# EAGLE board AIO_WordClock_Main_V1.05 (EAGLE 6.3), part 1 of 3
PROJECT_AUTHOR: Carsten Wille; PROJECT_COPYRIGHT: (c) 11/2012; PROJECT_NAME: WordClock; PROJECT_PCB_NO: PCB#201211001; PROJECT_REVISION: 1.05
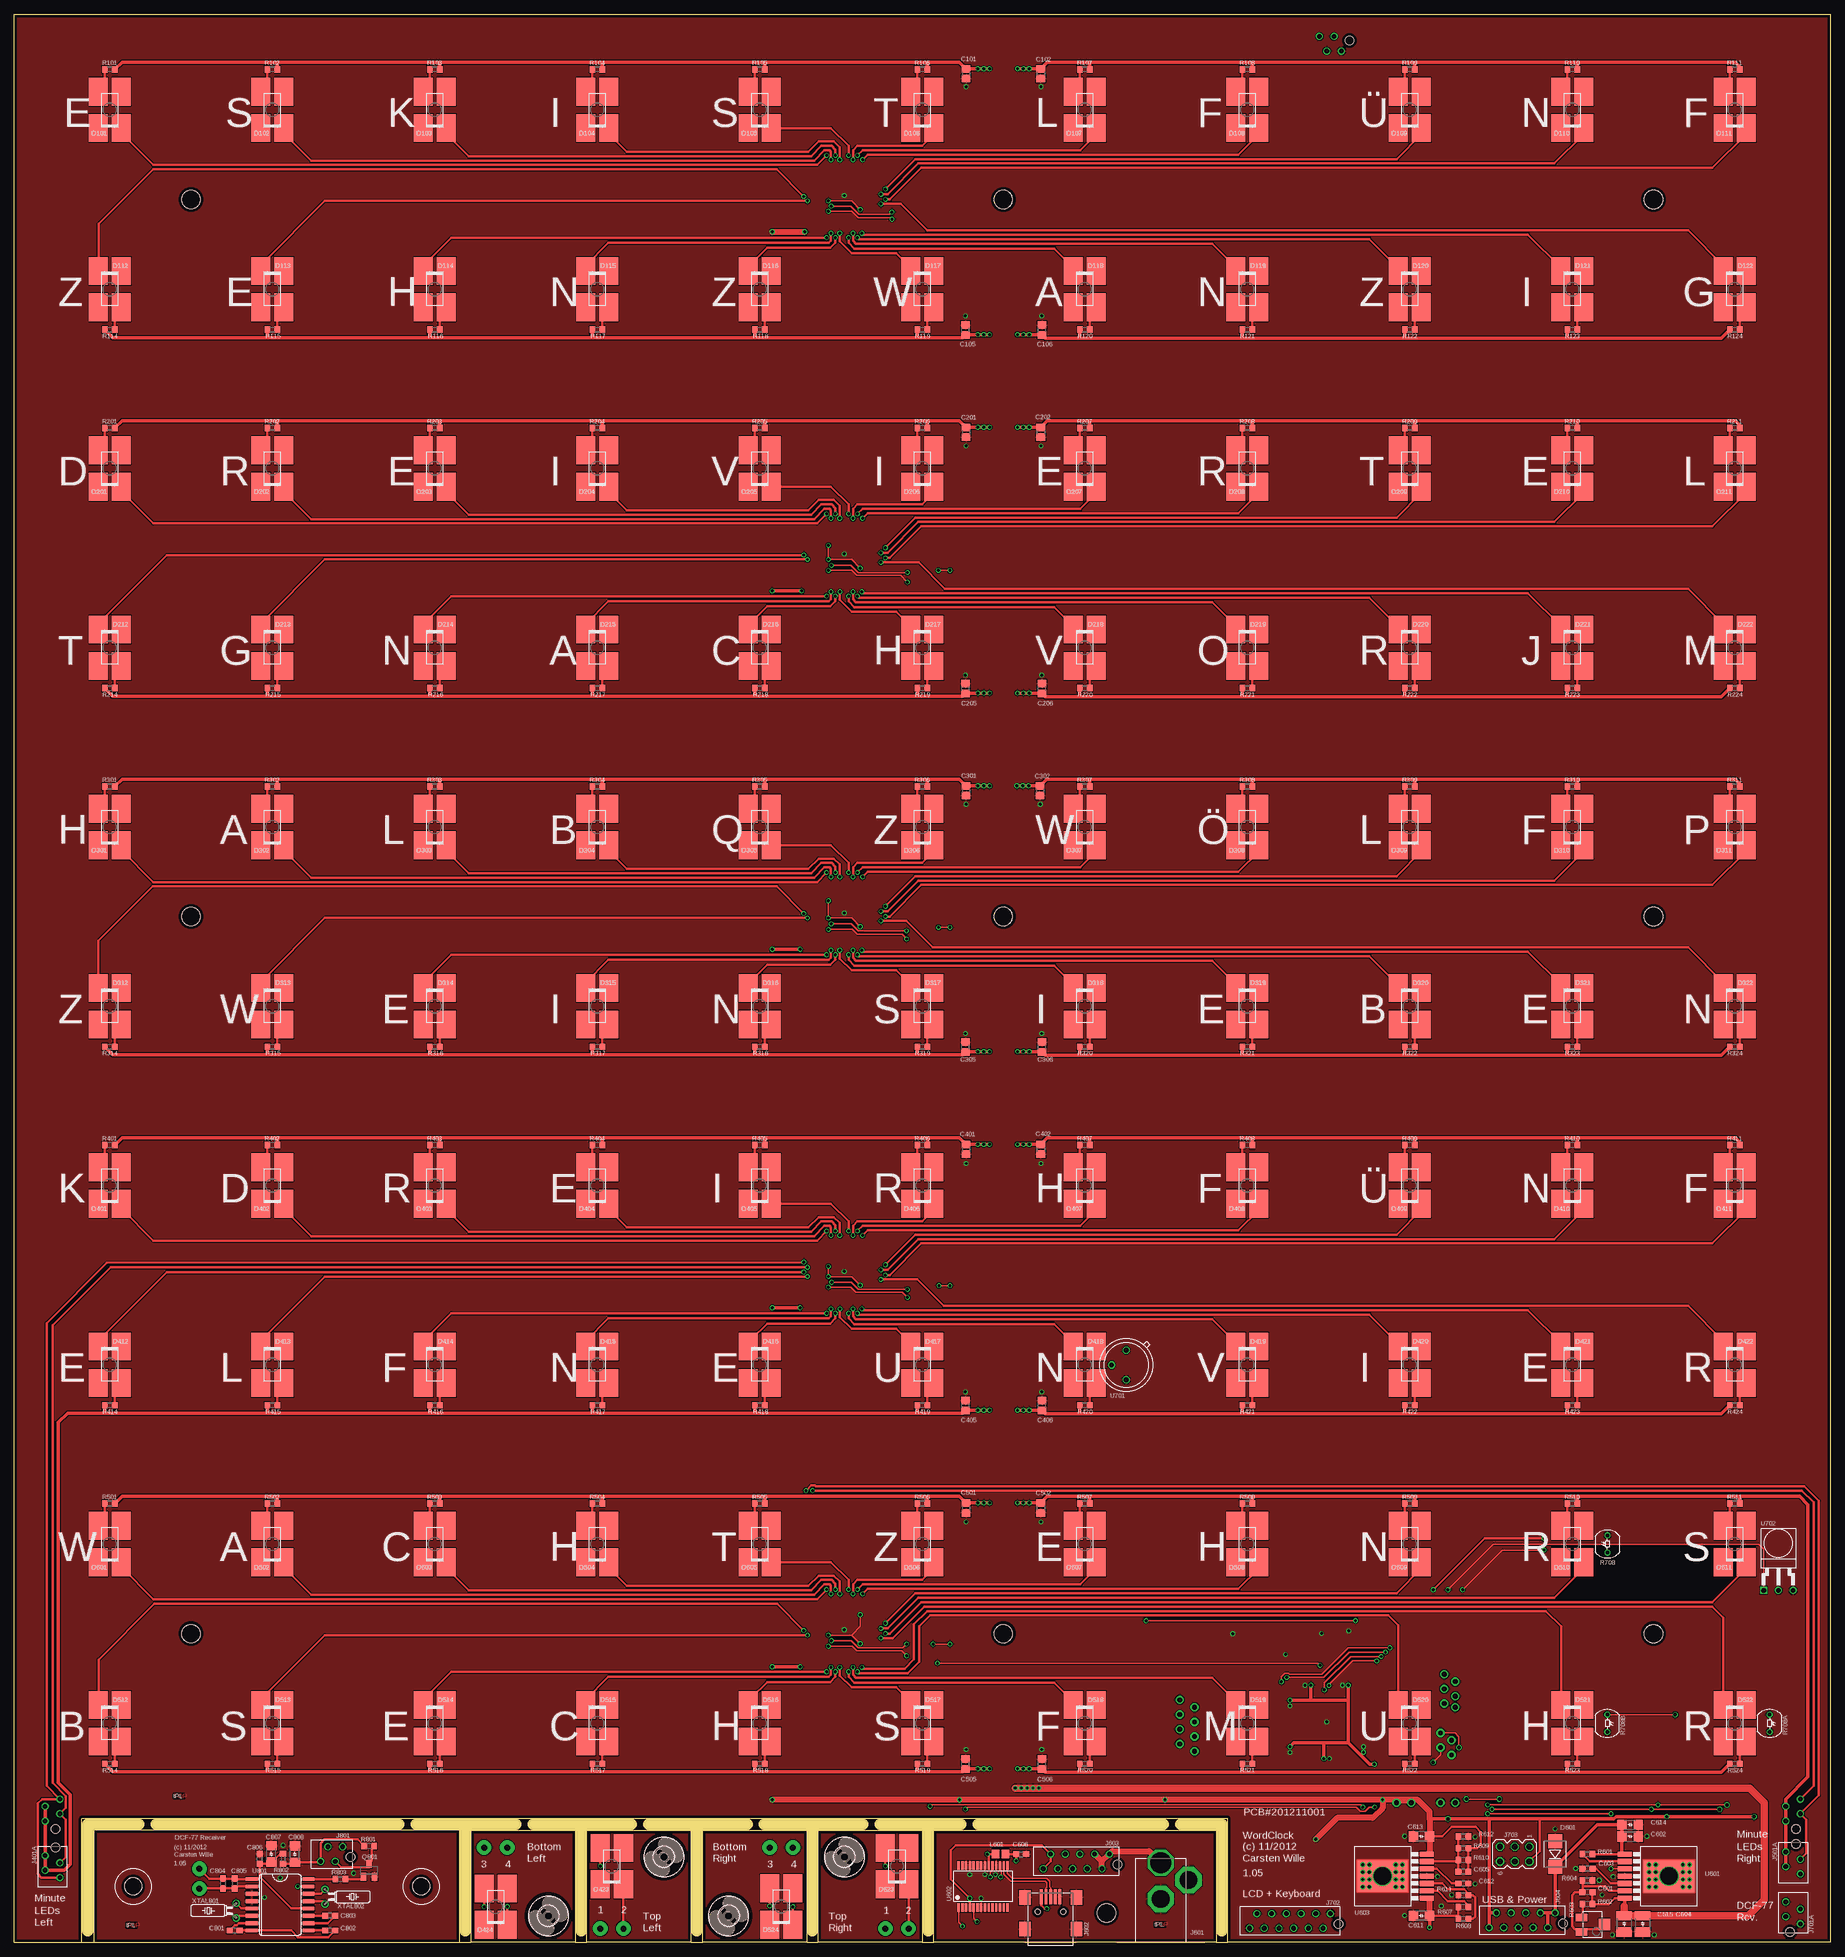
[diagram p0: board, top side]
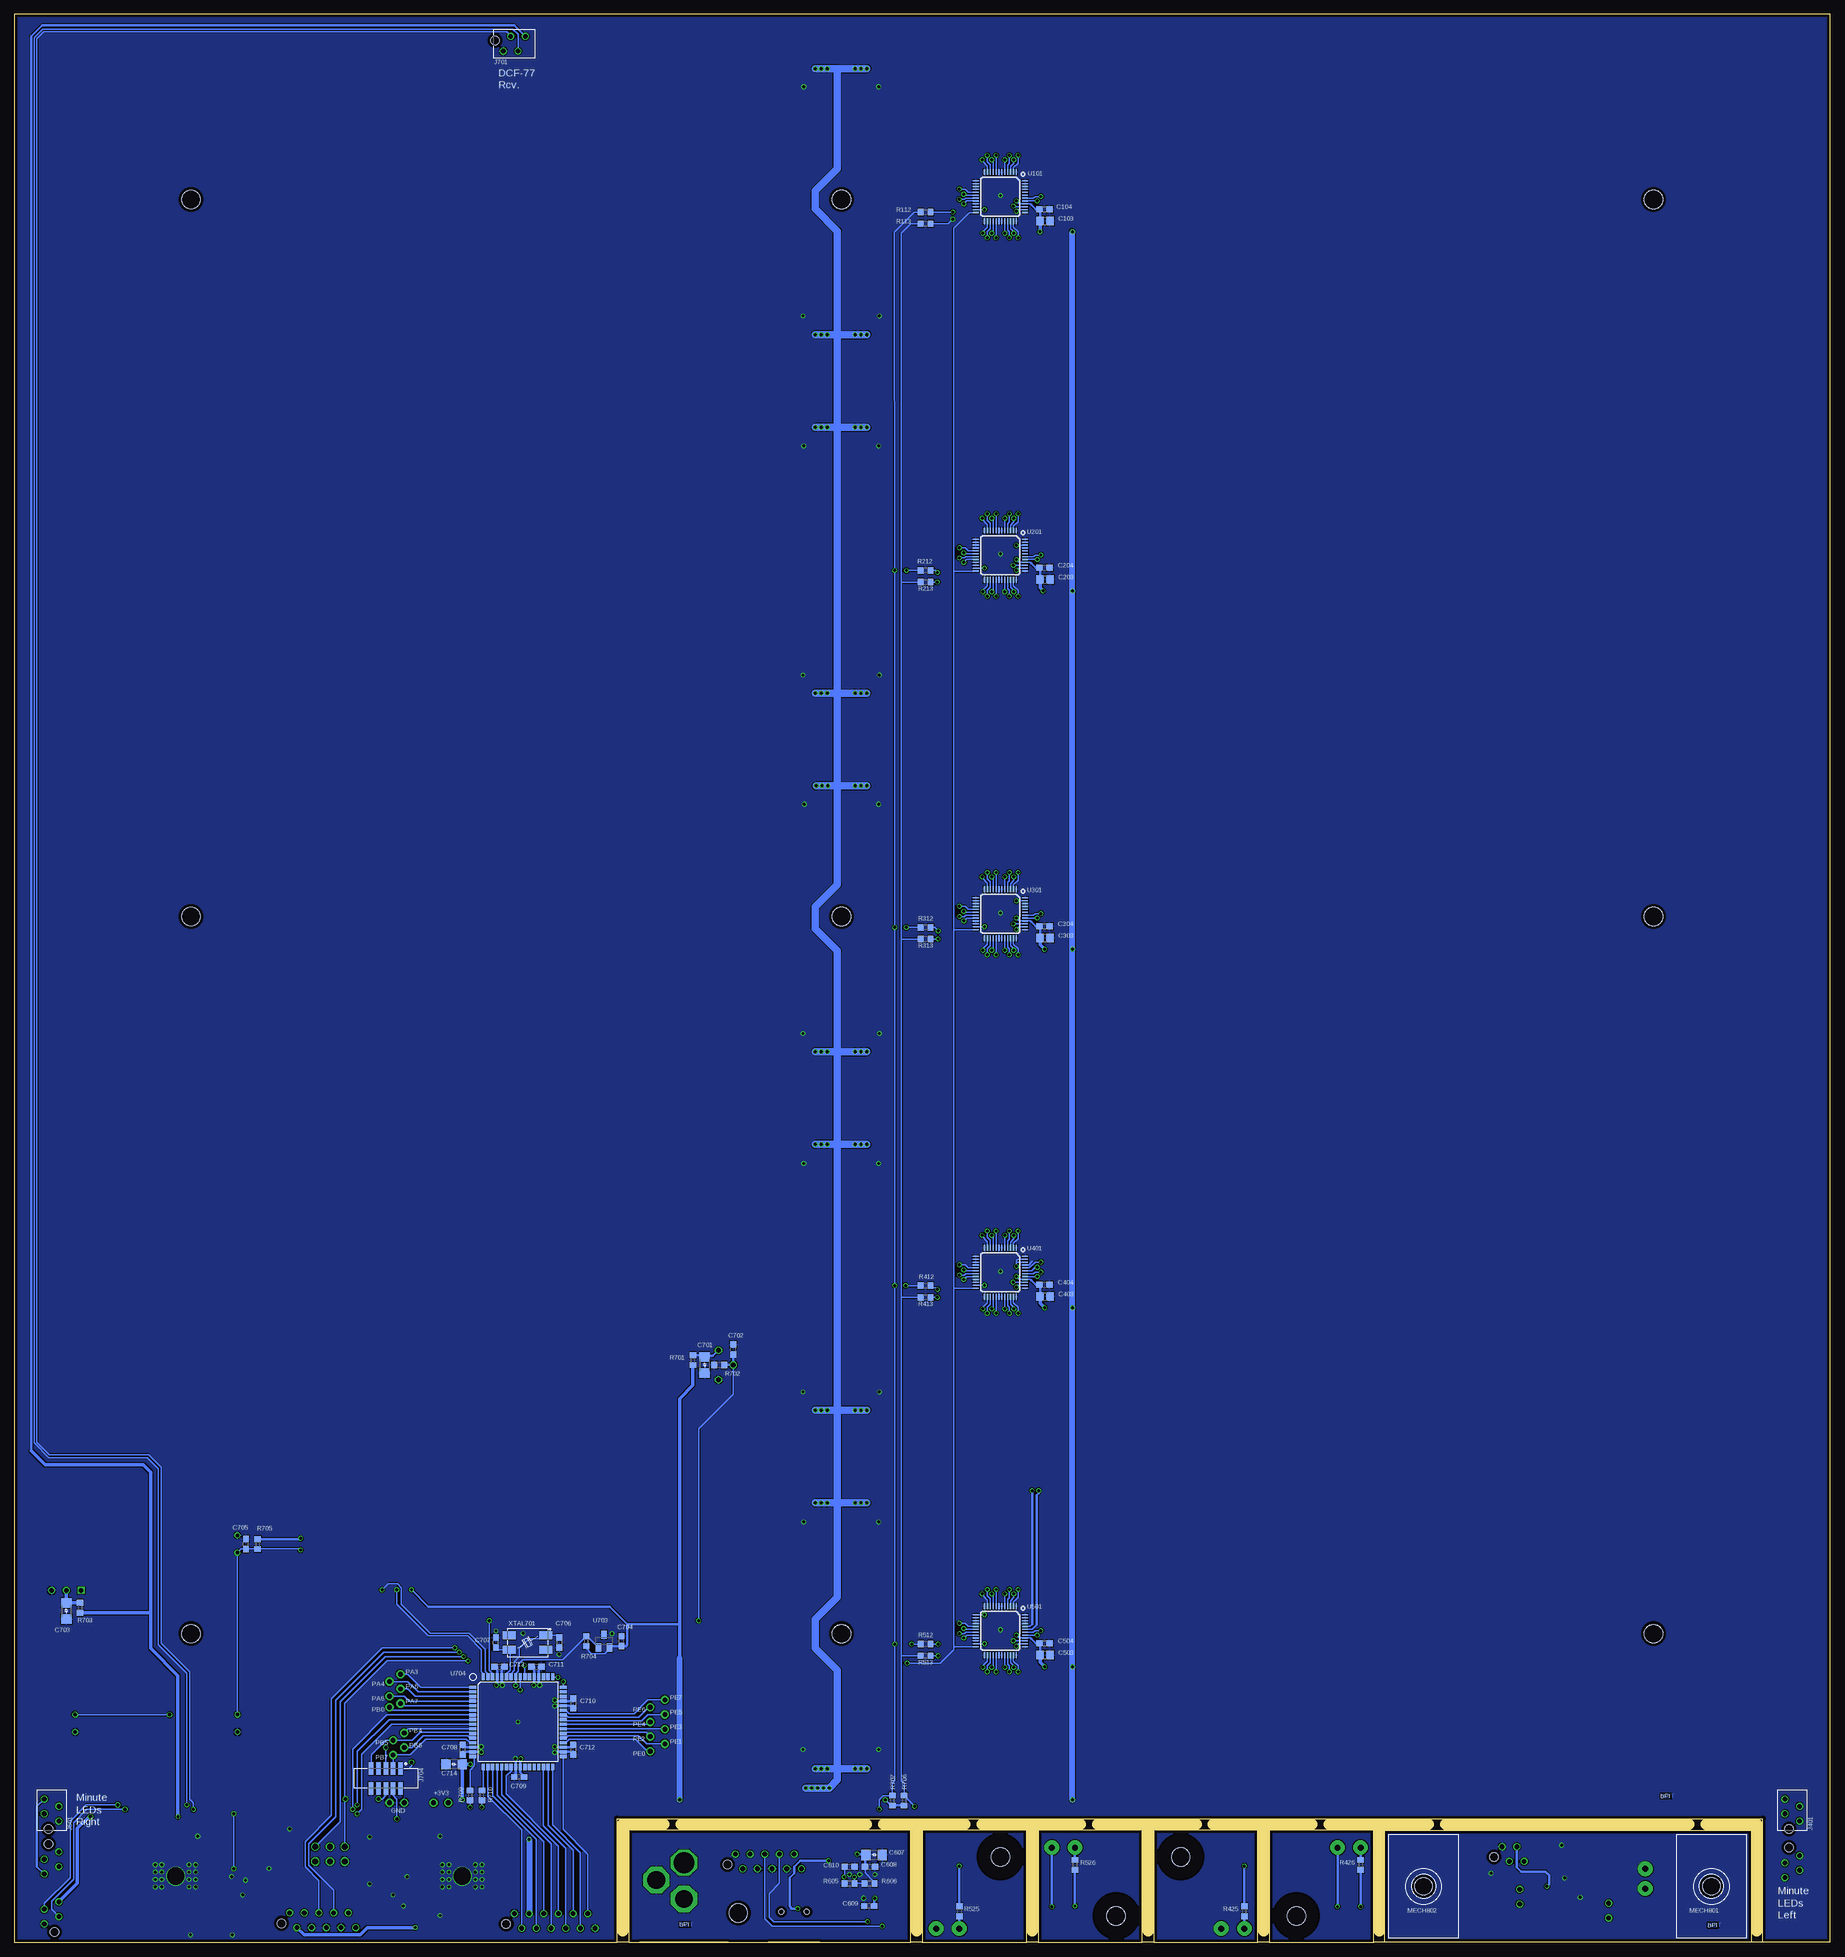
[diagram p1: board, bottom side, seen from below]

Size 314 x 333.4 mm. Coordinates in mm from the lower left corner, seen from the top.
Copper layers (1*16): Top 0.035mm / dielectric 1.5mm / Bottom 0.035mm
Design rules "leiton": minimum track width 6mil, minimum drill 12mil, track to track 6mil, track to pad 6mil, pad to pad 6mil, via to via 6mil, smd to smd 6mil, copper to edge 20mil, drill to drill 8mil, minimum pad ring 8mil, minimum via ring 6mil, stop-mask expansion 3mil, vias tented up to drill 0mil, thermal gap 8mil
Holes 3.2 mm at 188.82,5.12

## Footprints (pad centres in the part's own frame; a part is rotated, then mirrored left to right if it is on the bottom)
C0805 = smd 1.3 x 1.5: 1 -0.85,0; 2 0.85,0
C0603 = smd 1.1 x 1: 1 -0.85,0; 2 0.85,0
C1206 = smd 1.6 x 1.8: 1 -1.4,0; 2 1.4,0
C1210 = smd 1.6 x 2.7: 1 -1.4,0; 2 1.4,0
P-LCC-2 = smd 3.3 x 4.8: A -2,3.15; C 2,-3.15; NC@0 2,3.15; NC@1 -2,-3.15
SMB = smd 2.4 x 2.4: A 2.2,0; C -2.2,0
3,2 = hole 3.2: 0,0
MICRO-MATCH-4 = drill 0.8: 1 -1.905,-1.27; 2 -0.635,1.27; 3 0.635,-1.27; 4 1.905,1.27 | hole 1.5: -3.305,0.53
RAPC722X = drill 3.556 pad 4.572 octagon: 1 0,13.741 | drill 3.048 pad 4.572 octagon: 2 0,7.493; 3 4.801,10.744
USB-MINI-B-SMD = smd 2.6 x 0.5: 1 2.6,1.6; 2 2.6,0.8; 3 2.6,0; 4 2.6,-0.8; 5 2.6,-1.6 | smd 2.5 x 2: S0 -3,4.45; S1 2.5,4.45; S2 2.5,-4.45; S3 -3,-4.45 | hole 0.9: 0,2.2; 0,-2.2
MICRO-MATCH-10 = drill 0.8: 1 -5.715,-1.27; 2 -4.445,1.27; 3 -3.175,-1.27; 4 -1.905,1.27; 5 -0.635,-1.27; 6 0.635,1.27; 7 1.905,-1.27; 8 3.175,1.27; 9 4.445,-1.27; 10 5.715,1.27 | hole 1.5: -7.115,0.53
MICRO-MATCH-12 = drill 0.8: 1 -6.985,-1.27; 2 -5.715,1.27; 3 -4.445,-1.27; 4 -3.175,1.27; 5 -1.905,-1.27; 6 -0.635,1.27; 7 0.635,-1.27; 8 1.905,1.27; 9 3.175,-1.27; 10 4.445,1.27; 11 5.715,-1.27; 12 6.985,1.27 | hole 1.5: -8.385,0.53
MA03-2 = drill 1.016: 1 -1.27,2.54 | drill 1.016 octagon: 2 1.27,2.54; 3 -1.27,0; 4 1.27,0; 5 -1.27,-2.54; 6 1.27,-2.54
FTS-105-01-L-DV = smd 0.762 x 2.159: 1 -2.54,-1.714; 2 -2.54,1.714; 3 -1.27,-1.714; 4 -1.27,1.714; 5 0,-1.714; 6 0,1.714; 7 1.27,-1.714; 8 1.27,1.714; 9 2.54,-1.714; 10 2.54,1.714
L0805 = smd 1.3 x 1.5: 1 -0.85,0; 2 0.85,0
SOCKET = hole 3: 0,0
WORDCLOCK_S = hole 3.2: 281.95,30.5; 29.05,278.5; 29.05,30.5; 281.95,278.5; 29.05,154.5; 281.95,154.5; 169.5,30.5; 169.5,154.5; 169.5,278.5
SOT23 = smd 1 x 1.4: 1 -0.95,-1.1; 2 0.95,-1.1; 3 0,1.1
R0603 = smd 1 x 1.1: 1 -0.85,0; 2 0.85,0
RTRIM3224W = smd 1.3 x 2: 1 -1.25,-1.904; 3 1.25,-1.904 | smd 2 x 2: 2 0,2.031
LDR_A90 = drill 0.6: 1 -1.5,0; 2 1.5,0
LQFP48 = smd 0.203 x 1: 1 -2.75,-4.25; 2 -2.25,-4.25; 3 -1.75,-4.25; 4 -1.25,-4.25; 5 -0.75,-4.25; 6 -0.25,-4.25; 7 0.25,-4.25; 8 0.75,-4.25; 9 1.25,-4.25; 10 1.75,-4.25; 11 2.25,-4.25; 12 2.75,-4.25; 25 2.75,4.25; 26 2.25,4.25; 27 1.75,4.25; 28 1.25,4.25; 29 0.75,4.25; 30 0.25,4.25; 31 -0.25,4.25; 32 -0.75,4.25; 33 -1.25,4.25; 34 -1.75,4.25; 35 -2.25,4.25; 36 -2.75,4.25 | smd 1 x 0.203: 13 4.25,-2.75; 14 4.25,-2.25; 15 4.25,-1.75; 16 4.25,-1.25; 17 4.25,-0.75; 18 4.25,-0.25; 19 4.25,0.25; 20 4.25,0.75; 21 4.25,1.25; 22 4.25,1.75; 23 4.25,2.25; 24 4.25,2.75; 37 -4.25,2.75; 38 -4.25,2.25; 39 -4.25,1.75; 40 -4.25,1.25; 41 -4.25,0.75; 42 -4.25,0.25; 43 -4.25,-0.25; 44 -4.25,-0.75; 45 -4.25,-1.25; 46 -4.25,-1.75; 47 -4.25,-2.25; 48 -4.25,-2.75
TO-PMOD-7HS = smd 0.89 x 2.41: 1 -3.81,-7.63; 2 -2.54,-7.63; 3 -1.27,-7.63; 4 0,-7.63; 5 1.27,-7.63; 6 2.54,-7.63; 7 3.81,-7.63 | smd 5.35 x 8.54: HS 0,0
SSOP28 = smd 0.4 x 1.5: 1 -4.225,-3.625; 2 -3.575,-3.625; 3 -2.925,-3.625; 4 -2.275,-3.625; 5 -1.625,-3.625; 6 -0.975,-3.625; 7 -0.325,-3.625; 8 0.325,-3.625; 9 0.975,-3.625; 10 1.625,-3.625; 11 2.275,-3.625; 12 2.925,-3.625; 13 3.575,-3.625; 14 4.225,-3.625; 15 4.225,3.625; 16 3.575,3.625; 17 2.925,3.625; 18 2.275,3.625; 19 1.625,3.625; 20 0.975,3.625; 21 0.325,3.625; 22 -0.325,3.625; 23 -0.975,3.625; 24 -1.625,3.625; 25 -2.275,3.625; 26 -2.925,3.625; 27 -3.575,3.625; 28 -4.225,3.625
TO-5 = drill 0.813 octagon: 1 0,-2.54; 2 2.54,0; 3 0,2.54
TSOP322 = drill 0.8 square: 1 -2.54,-2.54 | drill 0.8: 2 0,-2.54; 3 2.54,-2.54
TQFP64 = smd 1.194 x 0.559: 1 -7.8,6; 2 -7.8,5.2; 3 -7.8,4.4; 4 -7.8,3.6; 5 -7.8,2.8; 6 -7.8,2; 7 -7.8,1.2; 8 -7.8,0.4; 9 -7.8,-0.4; 10 -7.8,-1.2; 11 -7.8,-2; 12 -7.8,-2.8; 13 -7.8,-3.6; 14 -7.8,-4.4; 15 -7.8,-5.2; 16 -7.8,-6; 33 7.8,-6; 34 7.8,-5.2; 35 7.8,-4.4; 36 7.8,-3.6; 37 7.8,-2.8; 38 7.8,-2; 39 7.8,-1.2; 40 7.8,-0.4; 41 7.8,0.4; 42 7.8,1.2; 43 7.8,2; 44 7.8,2.8; 45 7.8,3.6; 46 7.8,4.4; 47 7.8,5.2; 48 7.8,6 | smd 0.559 x 1.194: 17 -6,-7.8; 18 -5.2,-7.8; 19 -4.4,-7.8; 20 -3.6,-7.8; 21 -2.8,-7.8; 22 -2,-7.8; 23 -1.2,-7.8; 24 -0.4,-7.8; 25 0.4,-7.8; 26 1.2,-7.8; 27 2,-7.8; 28 2.8,-7.8; 29 3.6,-7.8; 30 4.4,-7.8; 31 5.2,-7.8; 32 6,-7.8; 49 6,7.8; 50 5.2,7.8; 51 4.4,7.8; 52 3.6,7.8; 53 2.8,7.8; 54 2,7.8; 55 1.2,7.8; 56 0.4,7.8; 57 -0.4,7.8; 58 -1.2,7.8; 59 -2,7.8; 60 -2.8,7.8; 61 -3.6,7.8; 62 -4.4,7.8; 63 -5.2,7.8; 64 -6,7.8
SO16L = smd 0.66 x 2.032: 1 -4.445,-4.902; 2 -3.175,-4.902; 3 -1.905,-4.902; 4 -0.635,-4.902; 5 0.635,-4.902; 6 1.905,-4.902; 7 3.175,-4.902; 8 4.445,-4.902; 9 4.445,4.902; 10 3.175,4.902; 11 1.905,4.902; 12 0.635,4.902; 13 -0.635,4.902; 14 -1.905,4.902; 15 -3.175,4.902; 16 -4.445,4.902
SINGLE-PIN = drill 0.813 pad 1.422: P$1 0,0
SINGLE-PIN_BIG = drill 1.016 pad 2.54: 1 0,0
MQ = smd 2.2 x 1.4: 1 -3.15,-1.25; 2 3.15,-1.25; 3 3.15,1.25; 4 -3.15,1.25
TC26H = drill 0.813: 1 -1.27,0; 2 1.27,0

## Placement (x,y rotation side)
C101  1E-6-1U-0805  [C0805]  164.57,323.15 270 top
C102  1E-6-1U-0805  [C0805]  177.46,323.15 270 top
C103  1E-6-1U-0805  [C0805]  135.81,297.7 0 bottom
C104  1E-9-100N-0603  [C0603]  135.88,299.73 0 bottom
C105  1E-6-1U-0805  [C0805]  164.47,278.84 90 top
C106  1E-6-1U-0805  [C0805]  177.69,278.84 90 top
C201  1E-6-1U-0805  [C0805]  164.57,261.15 270 top
C202  1E-6-1U-0805  [C0805]  177.46,261.15 270 top
C203  1E-6-1U-0805  [C0805]  135.81,235.7 0 bottom
C204  1E-9-100N-0603  [C0603]  135.88,237.73 0 bottom
C205  1E-6-1U-0805  [C0805]  164.47,216.84 90 top
C206  1E-6-1U-0805  [C0805]  177.69,216.84 90 top
C301  1E-6-1U-0805  [C0805]  164.57,199.15 270 top
C302  1E-6-1U-0805  [C0805]  177.33,199.15 270 top
C303  1E-6-1U-0805  [C0805]  135.81,173.7 0 bottom
C304  1E-9-100N-0603  [C0603]  135.88,175.73 0 bottom
C305  1E-6-1U-0805  [C0805]  164.47,154.84 90 top
C306  1E-6-1U-0805  [C0805]  177.69,154.84 90 top
C401  1E-6-1U-0805  [C0805]  164.57,137.15 270 top
C402  1E-6-1U-0805  [C0805]  177.46,137.15 270 top
C403  1E-6-1U-0805  [C0805]  135.81,111.7 0 bottom
C404  1E-9-100N-0603  [C0603]  135.88,113.73 0 bottom
C405  1E-6-1U-0805  [C0805]  164.47,92.84 90 top
C406  1E-6-1U-0805  [C0805]  177.69,92.84 90 top
C501  1E-6-1U-0805  [C0805]  164.57,75.15 270 top
C502  1E-6-1U-0805  [C0805]  177.46,75.15 270 top
C503  1E-6-1U-0805  [C0805]  135.81,49.7 0 bottom
C504  1E-9-100N-0603  [C0603]  135.88,51.73 0 bottom
C505  1E-6-1U-0805  [C0805]  164.47,30.84 90 top
C506  1E-6-1U-0805  [C0805]  177.69,30.84 90 top
C601  1E-9-22N-0603  [C0603]  272.01,8.68 180 top
C602  1E-6-10U-1206  [C1206]  279.38,18.33 0 top
C603  1E-9-22N-0603  [C0603]  272.01,12.74 180 top
C604  1E-6-47U-1210  [C1210]  281.54,3.21 270 top
C605  1E-9-22N-0603  [C0603]  250.55,12.23 180 top
C606  1E-9-10N-0603  [C0603]  174.09,15.28 0 top
C607  1E-6-10U-1206  [C1206]  165.33,15.15 0 bottom
C608  1E-9-100N-0603  [C0603]  166.07,13.07 0 bottom
C609  1E-9-100N-0603  [C0603]  166.19,6.31 180 bottom
C610  1E-9-100N-0603  [C0603]  169.57,13.07 0 bottom
C611  1E-6-10U-1206  [C1206]  243.31,4.61 180 top
C612  1E-9-22N-0603  [C0603]  250.55,10.2 0 top
C613  1E-6-10U-1206  [C1206]  243.31,18.33 180 top
C614  1E-6-10U-1206  [C1206]  279.38,20.36 0 top
C615  1E-6-47U-1210  [C1210]  278.36,3.21 270 top
C701  1E-6-10U-1206  [C1206]  194.67,99.86 270 bottom
C702  1E-9-33N-0603  [C0603]  189.71,102.53 90 bottom
C703  1E-6-10U-1206  [C1206]  305.03,57.32 270 bottom
C704  1E-9-100N-0603  [C0603]  209.02,52.11 90 bottom
C705  1E-9-33N-0603  [C0603]  273.97,68.9 90 bottom
C706  1E-12-22P-0603  [C0603]  219.81,51.86 270 bottom
C707  1E-12-22P-0603  [C0603]  230.74,51.86 90 bottom
C708  1E-9-100N-0603  [C0603]  236.48,33.34 90 bottom
C709  1E-9-100N-0603  [C0603]  226.72,28.61 180 bottom
C710  1E-9-100N-0603  [C0603]  217.37,41.34 270 bottom
C711  1E-9-100N-0603  [C0603]  223.72,47.69 0 bottom
C712  1E-9-100N-0603  [C0603]  217.37,33.34 270 bottom
C713  1E-9-100N-0603  [C0603]  230.13,47.69 0 bottom
C714  1E-6-10U-1206  [C1206]  237.97,30.82 180 bottom
C801  1E-9-6.8N-0603  [C0603]  38.08,2.07 0 top
C802  1E-9-33N-0603  [C0603]  54.59,2.07 180 top
C803  1E-9-10N-0603  [C0603]  54.59,4.61 180 top
C804  1E-9-1.5N-0603  [C0603]  36.04,10.2 270 top
C805  1E-9-1.5N-0603  [C0603]  38.08,10.2 270 top
C806  1E-9-100N-0603  [C0603]  42.39,14.47 90 top
C807  1E-6-10U-1206  [C1206]  44.43,15.31 90 top
C808  1E-6-10U-1206  [C1206]  48.49,15.28 90 top
D101  TOPLED-LUW  [P-LCC-2]  16.5,316.9 0 top
D102  TOPLED-LUW  [P-LCC-2]  44.6,316.9 0 top
D103  TOPLED-LUW  [P-LCC-2]  72.7,316.9 0 top
D104  TOPLED-LUW  [P-LCC-2]  100.8,316.9 0 top
D105  TOPLED-LUW  [P-LCC-2]  128.9,316.9 0 top
D106  TOPLED-LUW  [P-LCC-2]  157,316.9 0 top
D107  TOPLED-LUW  [P-LCC-2]  185.1,316.9 0 top
D108  TOPLED-LUW  [P-LCC-2]  213.2,316.9 0 top
D109  TOPLED-LUW  [P-LCC-2]  241.3,316.9 0 top
D110  TOPLED-LUW  [P-LCC-2]  269.4,316.9 0 top
D111  TOPLED-LUW  [P-LCC-2]  297.5,316.9 0 top
D112  TOPLED-LUW  [P-LCC-2]  16.5,285.9 180 top
D113  TOPLED-LUW  [P-LCC-2]  44.6,285.9 180 top
D114  TOPLED-LUW  [P-LCC-2]  72.7,285.9 180 top
D115  TOPLED-LUW  [P-LCC-2]  100.8,285.9 180 top
D116  TOPLED-LUW  [P-LCC-2]  128.9,285.9 180 top
D117  TOPLED-LUW  [P-LCC-2]  157,285.9 180 top
D118  TOPLED-LUW  [P-LCC-2]  185.1,285.9 180 top
D119  TOPLED-LUW  [P-LCC-2]  213.2,285.9 180 top
D120  TOPLED-LUW  [P-LCC-2]  241.3,285.9 180 top
D121  TOPLED-LUW  [P-LCC-2]  269.4,285.9 180 top
D122  TOPLED-LUW  [P-LCC-2]  297.5,285.9 180 top
D201  TOPLED-LUW  [P-LCC-2]  16.5,254.9 0 top
D202  TOPLED-LUW  [P-LCC-2]  44.6,254.9 0 top
D203  TOPLED-LUW  [P-LCC-2]  72.7,254.9 0 top
D204  TOPLED-LUW  [P-LCC-2]  100.8,254.9 0 top
D205  TOPLED-LUW  [P-LCC-2]  128.9,254.9 0 top
D206  TOPLED-LUW  [P-LCC-2]  157,254.9 0 top
D207  TOPLED-LUW  [P-LCC-2]  185.1,254.9 0 top
D208  TOPLED-LUW  [P-LCC-2]  213.2,254.9 0 top
D209  TOPLED-LUW  [P-LCC-2]  241.3,254.9 0 top
D210  TOPLED-LUW  [P-LCC-2]  269.4,254.9 0 top
D211  TOPLED-LUW  [P-LCC-2]  297.5,254.9 0 top
D212  TOPLED-LUW  [P-LCC-2]  16.5,223.9 180 top
D213  TOPLED-LUW  [P-LCC-2]  44.6,223.9 180 top
D214  TOPLED-LUW  [P-LCC-2]  72.7,223.9 180 top
D215  TOPLED-LUW  [P-LCC-2]  100.8,223.9 180 top
D216  TOPLED-LUW  [P-LCC-2]  128.9,223.9 180 top
D217  TOPLED-LUW  [P-LCC-2]  157,223.9 180 top
D218  TOPLED-LUW  [P-LCC-2]  185.1,223.9 180 top
D219  TOPLED-LUW  [P-LCC-2]  213.2,223.9 180 top
D220  TOPLED-LUW  [P-LCC-2]  241.3,223.9 180 top
D221  TOPLED-LUW  [P-LCC-2]  269.4,223.9 180 top
D222  TOPLED-LUW  [P-LCC-2]  297.5,223.9 180 top
D301  TOPLED-LUW  [P-LCC-2]  16.5,192.9 0 top
D302  TOPLED-LUW  [P-LCC-2]  44.6,192.9 0 top
D303  TOPLED-LUW  [P-LCC-2]  72.7,192.9 0 top
D304  TOPLED-LUW  [P-LCC-2]  100.8,192.9 0 top
D305  TOPLED-LUW  [P-LCC-2]  128.9,192.9 0 top
D306  TOPLED-LUW  [P-LCC-2]  157,192.9 0 top
D307  TOPLED-LUW  [P-LCC-2]  185.1,192.9 0 top
D308  TOPLED-LUW  [P-LCC-2]  213.2,192.9 0 top
D309  TOPLED-LUW  [P-LCC-2]  241.3,192.9 0 top
D310  TOPLED-LUW  [P-LCC-2]  269.4,192.9 0 top
D311  TOPLED-LUW  [P-LCC-2]  297.5,192.9 0 top
D312  TOPLED-LUW  [P-LCC-2]  16.5,161.9 180 top
D313  TOPLED-LUW  [P-LCC-2]  44.6,161.9 180 top
D314  TOPLED-LUW  [P-LCC-2]  72.7,161.9 180 top
D315  TOPLED-LUW  [P-LCC-2]  100.8,161.9 180 top
D316  TOPLED-LUW  [P-LCC-2]  128.9,161.9 180 top
D317  TOPLED-LUW  [P-LCC-2]  157,161.9 180 top
D318  TOPLED-LUW  [P-LCC-2]  185.1,161.9 180 top
D319  TOPLED-LUW  [P-LCC-2]  213.2,161.9 180 top
D320  TOPLED-LUW  [P-LCC-2]  241.3,161.9 180 top
D321  TOPLED-LUW  [P-LCC-2]  269.4,161.9 180 top
D322  TOPLED-LUW  [P-LCC-2]  297.5,161.9 180 top
D401  TOPLED-LUW  [P-LCC-2]  16.5,130.9 0 top
D402  TOPLED-LUW  [P-LCC-2]  44.6,130.9 0 top
D403  TOPLED-LUW  [P-LCC-2]  72.7,130.9 0 top
D404  TOPLED-LUW  [P-LCC-2]  100.8,130.9 0 top
D405  TOPLED-LUW  [P-LCC-2]  128.9,130.9 0 top
D406  TOPLED-LUW  [P-LCC-2]  157,130.9 0 top
D407  TOPLED-LUW  [P-LCC-2]  185.1,130.9 0 top
D408  TOPLED-LUW  [P-LCC-2]  213.2,130.9 0 top
D409  TOPLED-LUW  [P-LCC-2]  241.3,130.9 0 top
D410  TOPLED-LUW  [P-LCC-2]  269.4,130.9 0 top
D411  TOPLED-LUW  [P-LCC-2]  297.5,130.9 0 top
D412  TOPLED-LUW  [P-LCC-2]  16.5,99.9 180 top
D413  TOPLED-LUW  [P-LCC-2]  44.6,99.9 180 top
D414  TOPLED-LUW  [P-LCC-2]  72.7,99.9 180 top
D415  TOPLED-LUW  [P-LCC-2]  100.8,99.9 180 top
D416  TOPLED-LUW  [P-LCC-2]  128.9,99.9 180 top
D417  TOPLED-LUW  [P-LCC-2]  157,99.9 180 top
D418  TOPLED-LUW  [P-LCC-2]  185.1,99.9 180 top
D419  TOPLED-LUW  [P-LCC-2]  213.2,99.9 180 top
D420  TOPLED-LUW  [P-LCC-2]  241.3,99.9 180 top
D421  TOPLED-LUW  [P-LCC-2]  269.4,99.9 180 top
D422  TOPLED-LUW  [P-LCC-2]  297.5,99.9 180 top
D423  TOPLED-LUW  [P-LCC-2]  103.31,13.2 0 top
D424  TOPLED-LUW  [P-LCC-2]  83.21,6.2 0 top
D501  TOPLED-LUW  [P-LCC-2]  16.5,68.9 0 top
D502  TOPLED-LUW  [P-LCC-2]  44.6,68.9 0 top
D503  TOPLED-LUW  [P-LCC-2]  72.7,68.9 0 top
D504  TOPLED-LUW  [P-LCC-2]  100.8,68.9 0 top
D505  TOPLED-LUW  [P-LCC-2]  128.9,68.9 0 top
D506  TOPLED-LUW  [P-LCC-2]  157,68.9 0 top
D507  TOPLED-LUW  [P-LCC-2]  185.1,68.9 0 top
D508  TOPLED-LUW  [P-LCC-2]  213.2,68.9 0 top
D509  TOPLED-LUW  [P-LCC-2]  241.3,68.9 0 top
D510  TOPLED-LUW  [P-LCC-2]  269.4,68.9 0 top
D511  TOPLED-LUW  [P-LCC-2]  297.5,68.9 0 top
D512  TOPLED-LUW  [P-LCC-2]  16.5,37.9 180 top
D513  TOPLED-LUW  [P-LCC-2]  44.6,37.9 180 top
D514  TOPLED-LUW  [P-LCC-2]  72.7,37.9 180 top
D515  TOPLED-LUW  [P-LCC-2]  100.8,37.9 180 top
D516  TOPLED-LUW  [P-LCC-2]  128.9,37.9 180 top
D517  TOPLED-LUW  [P-LCC-2]  157,37.9 180 top
D518  TOPLED-LUW  [P-LCC-2]  185.1,37.9 180 top
D519  TOPLED-LUW  [P-LCC-2]  213.2,37.9 180 top
D520  TOPLED-LUW  [P-LCC-2]  241.3,37.9 180 top
D521  TOPLED-LUW  [P-LCC-2]  269.4,37.9 180 top
D522  TOPLED-LUW  [P-LCC-2]  297.5,37.9 180 top
D523  TOPLED-LUW  [P-LCC-2]  152.61,13.2 0 top
D524  TOPLED-LUW  [P-LCC-2]  132.6,6.22 0 top
D601  20BQ030-SMB  [SMB]  266.42,15.28 90 top
H401  MOUNT-HOLE3.2  [3,2]  92.31,4.6 0 top
H402  MOUNT-HOLE3.2  [3,2]  112.31,14.8 0 top
H501  MOUNT-HOLE3.2  [3,2]  123.51,4.6 0 top
H502  MOUNT-HOLE3.2  [3,2]  143.51,14.8 0 top
J401  MICRO-MATCH-4  [MICRO-MATCH-4]  6.58,22.9 90 bottom
J401A  MICRO-MATCH-4  [MICRO-MATCH-4]  6.58,13.12 270 top
J501  MICRO-MATCH-4  [MICRO-MATCH-4]  307.57,22.9 90 bottom
J501A  MICRO-MATCH-4  [MICRO-MATCH-4]  307.57,13.76 270 top
J601  PWR-JACK  [RAPC722X]  198.22,0.04 0 top
J602  USB_B_MINI  [USB-MINI-B-SMD]  179.17,5.3 90 top
J603  MICRO-MATCH-10  [MICRO-MATCH-10]  183.62,14.01 180 top
J604  MICRO-MATCH-10  [MICRO-MATCH-10]  260.71,3.85 180 top
J701  MICRO-MATCH-4  [MICRO-MATCH-4]  227.56,328.33 0 bottom
J701A  MICRO-MATCH-4  [MICRO-MATCH-4]  307.57,5.12 90 top
J702  MICRO-MATCH-12  [MICRO-MATCH-12]  220.57,3.72 180 top
J703  PROG-PDI  [MA03-2]  259.44,15.28 270 top
J704  JTAG_ATMEL-50MIL  [FTS-105-01-L-DV]  249.78,28.36 180 bottom
J801  MICRO-MATCH-4  [MICRO-MATCH-4]  54.84,15.28 180 top
L601  L-1U0-0805  [L0805]  170.54,15.28 180 top
MECH801  SOCKET  [SOCKET]  20.55,9.69 0 bottom
MECH802  SOCKET  [SOCKET]  70.33,9.69 0 bottom
PCB1  PCB-WORDCLOCK-ALL-IN-ONE  [WORDCLOCK_S]  1.5,22.9 0 top
Q801  BC847  [SOT23]  61.32,12.49 0 top
R101  1E0-3,0R-0603  [R0603]  16.5,323.9 180 top
R102  1E0-3,0R-0603  [R0603]  44.6,323.9 180 top
R103  1E0-3,0R-0603  [R0603]  72.7,323.9 180 top
R104  1E0-3,0R-0603  [R0603]  100.8,323.9 180 top
R105  1E0-3,0R-0603  [R0603]  128.9,323.9 180 top
R106  1E0-3,0R-0603  [R0603]  157,323.9 180 top
R107  1E0-3,0R-0603  [R0603]  185.1,323.9 180 top
R108  1E0-3,0R-0603  [R0603]  213.2,323.9 180 top
R109  1E0-3,0R-0603  [R0603]  241.3,323.9 180 top
R110  1E0-3,0R-0603  [R0603]  269.4,323.9 180 top
R111  1E0-3,0R-0603  [R0603]  297.5,323.9 180 top
R112  1E2-330R-0603  [R0603]  156.44,299.23 0 bottom
R113  1E2-330R-0603  [R0603]  156.44,297.22 0 bottom
R114  1E0-3,0R-0603  [R0603]  16.5,278.9 180 top
R115  1E0-3,0R-0603  [R0603]  44.6,278.9 180 top
R116  1E0-3,0R-0603  [R0603]  72.7,278.9 180 top
R117  1E0-3,0R-0603  [R0603]  100.8,278.9 180 top
R118  1E0-3,0R-0603  [R0603]  128.9,278.9 180 top
R119  1E0-3,0R-0603  [R0603]  157,278.9 180 top
R120  1E0-3,0R-0603  [R0603]  185.1,278.9 180 top
R121  1E0-3,0R-0603  [R0603]  213.2,278.9 180 top
R122  1E0-3,0R-0603  [R0603]  241.3,278.9 180 top
R123  1E0-3,0R-0603  [R0603]  269.4,278.9 180 top
R124  1E0-3,0R-0603  [R0603]  297.5,278.9 180 top
R201  1E0-3,0R-0603  [R0603]  16.5,261.9 180 top
R202  1E0-3,0R-0603  [R0603]  44.6,261.9 180 top
R203  1E0-3,0R-0603  [R0603]  72.7,261.9 180 top
R204  1E0-3,0R-0603  [R0603]  100.8,261.9 180 top
R205  1E0-3,0R-0603  [R0603]  128.9,261.9 180 top
R206  1E0-3,0R-0603  [R0603]  157,261.9 180 top
R207  1E0-3,0R-0603  [R0603]  185.1,261.9 180 top
R208  1E0-3,0R-0603  [R0603]  213.2,261.9 180 top
R209  1E0-3,0R-0603  [R0603]  241.3,261.9 180 top
R210  1E0-3,0R-0603  [R0603]  269.4,261.9 180 top
R211  1E0-3,0R-0603  [R0603]  297.5,261.9 180 top
R212  1E2-330R-0603  [R0603]  156.44,237.28 0 bottom
R213  1E2-330R-0603  [R0603]  156.44,235.24 0 bottom
R214  1E0-3,0R-0603  [R0603]  16.5,216.9 180 top
R215  1E0-3,0R-0603  [R0603]  44.6,216.9 180 top
R216  1E0-3,0R-0603  [R0603]  72.7,216.9 180 top
R217  1E0-3,0R-0603  [R0603]  100.8,216.9 180 top
R218  1E0-3,0R-0603  [R0603]  128.9,216.9 180 top
R219  1E0-3,0R-0603  [R0603]  157,216.9 180 top
R220  1E0-3,0R-0603  [R0603]  185.1,216.9 180 top
R221  1E0-3,0R-0603  [R0603]  213.2,216.9 180 top
R222  1E0-3,0R-0603  [R0603]  241.3,216.9 180 top
R223  1E0-3,0R-0603  [R0603]  269.4,216.9 180 top
R224  1E0-3,0R-0603  [R0603]  297.5,216.9 180 top
R301  1E0-3,0R-0603  [R0603]  16.5,199.9 180 top
R302  1E0-3,0R-0603  [R0603]  44.6,199.9 180 top
R303  1E0-3,0R-0603  [R0603]  72.7,199.9 180 top
R304  1E0-3,0R-0603  [R0603]  100.8,199.9 180 top
R305  1E0-3,0R-0603  [R0603]  128.9,199.9 180 top
R306  1E0-3,0R-0603  [R0603]  157,199.9 180 top
R307  1E0-3,0R-0603  [R0603]  185.1,199.9 180 top
R308  1E0-3,0R-0603  [R0603]  213.2,199.9 180 top
R309  1E0-3,0R-0603  [R0603]  241.3,199.9 180 top
R310  1E0-3,0R-0603  [R0603]  269.4,199.9 180 top
R311  1E0-3,0R-0603  [R0603]  297.5,199.9 180 top
R312  1E2-330R-0603  [R0603]  156.44,175.53 0 bottom
R313  1E2-330R-0603  [R0603]  156.44,173.52 0 bottom
R314  1E0-3,0R-0603  [R0603]  16.5,154.9 180 top
R315  1E0-3,0R-0603  [R0603]  44.6,154.9 180 top
R316  1E0-3,0R-0603  [R0603]  72.7,154.9 180 top
R317  1E0-3,0R-0603  [R0603]  100.8,154.9 180 top
R318  1E0-3,0R-0603  [R0603]  128.9,154.9 180 top
R319  1E0-3,0R-0603  [R0603]  157,154.9 180 top
R320  1E0-3,0R-0603  [R0603]  185.1,154.9 180 top
R321  1E0-3,0R-0603  [R0603]  213.2,154.9 180 top
R322  1E0-3,0R-0603  [R0603]  241.3,154.9 180 top
R323  1E0-3,0R-0603  [R0603]  269.4,154.9 180 top
R324  1E0-3,0R-0603  [R0603]  297.5,154.9 180 top
R401  1E0-3,0R-0603  [R0603]  16.5,137.9 180 top
R402  1E0-3,0R-0603  [R0603]  44.6,137.9 180 top
R403  1E0-3,0R-0603  [R0603]  72.7,137.9 180 top
R404  1E0-3,0R-0603  [R0603]  100.8,137.9 180 top
R405  1E0-3,0R-0603  [R0603]  128.9,137.9 180 top
R406  1E0-3,0R-0603  [R0603]  157,137.9 180 top
R407  1E0-3,0R-0603  [R0603]  185.1,137.9 180 top
R408  1E0-3,0R-0603  [R0603]  213.2,137.9 180 top
R409  1E0-3,0R-0603  [R0603]  241.3,137.9 180 top
R410  1E0-3,0R-0603  [R0603]  269.4,137.9 180 top
R411  1E0-3,0R-0603  [R0603]  297.5,137.9 180 top
R412  1E2-330R-0603  [R0603]  156.44,113.58 0 bottom
R413  1E2-330R-0603  [R0603]  156.44,111.55 0 bottom
R414  1E0-3,0R-0603  [R0603]  16.5,92.9 180 top
R415  1E0-3,0R-0603  [R0603]  44.6,92.9 180 top
R416  1E0-3,0R-0603  [R0603]  72.7,92.9 180 top
R417  1E0-3,0R-0603  [R0603]  100.8,92.9 180 top
R418  1E0-3,0R-0603  [R0603]  128.9,92.9 180 top
R419  1E0-3,0R-0603  [R0603]  157,92.9 180 top
R420  1E0-3,0R-0603  [R0603]  185.1,92.9 180 top
R421  1E0-3,0R-0603  [R0603]  213.2,92.9 180 top
R422  1E0-3,0R-0603  [R0603]  241.3,92.9 180 top
R423  1E0-3,0R-0603  [R0603]  269.4,92.9 180 top
R424  1E0-3,0R-0603  [R0603]  297.5,92.9 180 top
R425  1E0-3,0R-0603  [R0603]  101.31,5.4 90 bottom
R426  1E0-3,0R-0603  [R0603]  81.21,13.4 270 bottom
R501  1E0-3,0R-0603  [R0603]  16.5,75.9 180 top
R502  1E0-3,0R-0603  [R0603]  44.6,75.9 180 top
R503  1E0-3,0R-0603  [R0603]  72.7,75.9 180 top
R504  1E0-3,0R-0603  [R0603]  100.8,75.9 180 top
R505  1E0-3,0R-0603  [R0603]  128.9,75.9 180 top
R506  1E0-3,0R-0603  [R0603]  157,75.9 180 top
R507  1E0-3,0R-0603  [R0603]  185.1,75.9 180 top
R508  1E0-3,0R-0603  [R0603]  213.2,75.9 180 top
R509  1E0-3,0R-0603  [R0603]  241.3,75.9 180 top
R510  1E0-3,0R-0603  [R0603]  269.4,75.9 180 top
R511  1E0-3,0R-0603  [R0603]  297.5,75.9 180 top
R512  1E2-330R-0603  [R0603]  156.44,51.6 0 bottom
R513  1E2-330R-0603  [R0603]  156.44,49.57 0 bottom
R514  1E0-3,0R-0603  [R0603]  16.5,30.9 180 top
R515  1E0-3,0R-0603  [R0603]  44.6,30.9 180 top
R516  1E0-3,0R-0603  [R0603]  72.7,30.9 180 top
R517  1E0-3,0R-0603  [R0603]  100.8,30.9 180 top
R518  1E0-3,0R-0603  [R0603]  128.9,30.9 180 top
R519  1E0-3,0R-0603  [R0603]  157,30.9 180 top
R520  1E0-3,0R-0603  [R0603]  185.1,30.9 180 top
R521  1E0-3,0R-0603  [R0603]  213.2,30.9 180 top
R522  1E0-3,0R-0603  [R0603]  241.3,30.9 180 top
R523  1E0-3,0R-0603  [R0603]  269.4,30.9 180 top
R524  1E0-3,0R-0603  [R0603]  297.5,30.9 180 top
R525  1E0-3,0R-0603  [R0603]  150.59,5.39 90 bottom
R526  1E0-3,0R-0603  [R0603]  130.61,13.4 270 bottom
R601  1E4-56K-0603  [R0603]  272.01,15.28 180 top
R602  1E3-3,3K-0603  [R0603]  272.01,6.64 180 top
R603  R-TRIM1K-3224W  [RTRIM3224W]  272.9,3.09 270 top
R604  1E3-1,1K-0603  [R0603]  272.01,10.71 0 top
R605  1E4-10K-0603  [R0603]  169.57,10.2 0 bottom
R606  1E3-4,7K-0603  [R0603]  166.12,10.2 180 bottom
R607  1E4-47K-0603  [R0603]  250.55,6.14 0 top
R608  1E4-33K-0603  [R0603]  250.55,4.1 0 top
R609  1E4-13K-0603  [R0603]  250.55,16.3 180 top
R610  1E3-4,7K-0603  [R0603]  250.55,14.26 180 top
R611  1E4-12K-0603  [R0603]  250.55,8.17 180 top
R612  1E3-1,1K-0603  [R0603]  250.55,18.33 0 top
R701  1E2-100R-0603  [R0603]  196.67,100.7 90 bottom
R702  1E4-47K-0603  [R0603]  192.13,99.86 180 bottom
R703  1E2-100R-0603  [R0603]  302.64,57.88 90 bottom
R704  1E4-10K-0603  [R0603]  215.11,52.11 90 bottom
R705  1E4-10K-0603  [R0603]  271.96,68.9 270 bottom
R706  1E3-3,3K-0603  [R0603]  160.15,24.55 90 bottom
R707  1E3-3,3K-0603  [R0603]  162.18,24.55 90 bottom
R708  LDR  [LDR_A90]  275.46,68.9 90 top
R708A  LDR  [LDR_A90]  303.51,37.89 270 top
R708B  LDR  [LDR_A90]  275.44,37.89 270 top
R709  1E2-330R-0603  [R0603]  235.21,25.44 90 bottom
R710  1E2-330R-0603  [R0603]  233.17,25.44 90 bottom
R801  1E4-10K-0603  [R0603]  61.32,16.68 0 top
R802  1E2-100R-0603  [R0603]  46.46,14.47 270 top
R803  1E5-100K-0603  [R0603]  56.36,10.96 0 top
U101  PCA9626  [LQFP48]  143.5,301.9 180 bottom
U201  PCA9626  [LQFP48]  143.5,239.9 180 bottom
U301  PCA9626  [LQFP48]  143.5,177.9 180 bottom
U401  PCA9626  [LQFP48]  143.5,115.9 180 bottom
U501  PCA9626  [LQFP48]  143.5,53.9 180 bottom
U601  LMZ12003  [TO-PMOD-7HS]  286.11,11.47 270 top
U602  FT232RL  [SSOP28]  167.49,9.69 0 top
U603  LMZ12003  [TO-PMOD-7HS]  236.58,11.47 90 top
U701  LHI1128  [TO-5]  192.25,99.86 180 top
U702  TSOP32236  [TSOP322]  305.03,63.41 0 top
U703  MCP120  [SOT23]  212.07,52.11 0 bottom
U704  XMEGA64A3  [TQFP64]  226.93,38.14 0 bottom
U801  U4224B  [SO16L]  45.95,6.52 270 top
X1  SINGLE-PIN-36MIL  [SINGLE-PIN]  204.06,33.06 180 top
X2  SINGLE-PIN-36MIL  [SINGLE-PIN]  201.53,34.33 180 top
X3  SINGLE-PIN-36MIL  [SINGLE-PIN]  204.06,35.6 180 top
X4  SINGLE-PIN-36MIL  [SINGLE-PIN]  201.53,36.87 180 top
X5  SINGLE-PIN-36MIL  [SINGLE-PIN]  204.06,38.14 180 top
X6  SINGLE-PIN-36MIL  [SINGLE-PIN]  201.53,39.41 180 top
X7  SINGLE-PIN-36MIL  [SINGLE-PIN]  204.06,40.68 180 top
X8  SINGLE-PIN-36MIL  [SINGLE-PIN]  201.53,41.95 180 top
X9  SINGLE-PIN-36MIL  [SINGLE-PIN]  247.25,46.39 0 top
X10  SINGLE-PIN-36MIL  [SINGLE-PIN]  249.15,45.12 0 top
X11  SINGLE-PIN-36MIL  [SINGLE-PIN]  247.25,43.85 0 top
X12  SINGLE-PIN-36MIL  [SINGLE-PIN]  249.15,42.58 0 top
X13  SINGLE-PIN-36MIL  [SINGLE-PIN]  247.25,41.31 0 top
X14  SINGLE-PIN-36MIL  [SINGLE-PIN]  249.15,40.68 0 top
X15  SINGLE-PIN-36MIL  [SINGLE-PIN]  246.61,36.23 0 top
X16  SINGLE-PIN-36MIL  [SINGLE-PIN]  248.51,34.96 0 top
X17  SINGLE-PIN-36MIL  [SINGLE-PIN]  246.61,33.7 0 top
X18  SINGLE-PIN-36MIL  [SINGLE-PIN]  248.51,32.42 0 top
X21  SINGLE-PIN-36MIL  [SINGLE-PIN]  246.61,24.17 90 top
X22  SINGLE-PIN-36MIL  [SINGLE-PIN]  249.15,24.17 90 top
X23  SINGLE-PIN-36MIL  [SINGLE-PIN]  241.53,24.17 90 top
X24  SINGLE-PIN-36MIL  [SINGLE-PIN]  238.99,24.17 90 top
X401  SINGLE-PIN-40MIL  [SINGLE-PIN_BIG]  101.31,2.4 90 top
X402  SINGLE-PIN-40MIL  [SINGLE-PIN_BIG]  81.21,16.4 90 top
X403  SINGLE-PIN-40MIL  [SINGLE-PIN_BIG]  105.31,2.4 90 top
X404  SINGLE-PIN-40MIL  [SINGLE-PIN_BIG]  85.21,16.4 90 top
X501  SINGLE-PIN-40MIL  [SINGLE-PIN_BIG]  150.61,2.4 90 top
X502  SINGLE-PIN-40MIL  [SINGLE-PIN_BIG]  130.61,16.4 90 top
X503  SINGLE-PIN-40MIL  [SINGLE-PIN_BIG]  154.61,2.4 90 top
X504  SINGLE-PIN-40MIL  [SINGLE-PIN_BIG]  134.61,16.4 90 top
X801  SINGLE-PIN-40MIL  [SINGLE-PIN_BIG]  31.98,12.74 270 top
X802  SINGLE-PIN-40MIL  [SINGLE-PIN_BIG]  31.98,9.31 270 top
XTAL701  MQ-8.000  [MQ]  225.27,51.86 180 bottom
XTAL801  TC26-77.5  [TC26H]  38.33,5.5 90 top
XTAL802  TC26-77.5  [TC26H]  53.7,7.91 270 top

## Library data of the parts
C101-C103 C105 C106 C201-C203 C205 C206 C301-C303 C305 C306 C401-C403 C405 C406 C501-C503 C505 C506 = o.Capacitor 0603 0805 1206; MATERIAL: X7R; ORDER-MULTIPLE: 10; PACKAGE: 0805; SUPPLIER: Farnell; SUPPLIER-NUMBER: 145-8903; TOLERANCE: 10%; VAL: 1µ; VENDOR: Phycomp; VENDOR-NUMBER: 222291015663; VOLTAGE: 25V
C104 C204 C304 C404 C504 C608-C610 C704 C708-C713 C806 = o.Capacitor 0603 0805 1206; MATERIAL: X7R; ORDER-MULTIPLE: 10; SUPPLIER: Farnell; SUPPLIER-NUMBER: 882-0023; TOLERANCE: 10%; VAL: 100n; VENDOR: Murata; VENDOR-NUMBER: GRM188R71H104KA93D; VOLTAGE: 50V
C601 C603 C605 C612 = o.Capacitor 0603 0805 1206; MATERIAL: X7R; ORDER-MULTIPLE: 10; SUPPLIER: Farnell; SUPPLIER-NUMBER: 141-4626; TOLERANCE: 10%; VAL: 220n; VENDOR: Kemet; VENDOR-NUMBER: C0603C224K3RAC; VOLTAGE: 25V
C602 C607 C611 C613 C701 C703 C714 C807 C808 = o.Capacitor 0603 0805 1206; MATERIAL: X7R; ORDER-MULTIPLE: 1; PACKAGE: 1206; SUPPLIER: Reichelt; SUPPLIER-NUMBER: X5R-G1206 10/25; TOLERANCE: 10%; VAL: 10µ; VOLTAGE: 25V
C604 C615 = o.Capacitor 0603 0805 1206.v6; MATERIAL: Y5V; ORDER-MULTIPLE: 10; PACKAGE: 1210; SUPPLIER: Farnell; SUPPLIER-NUMBER: 1759367; TOLERANCE: +80%/-20%; VAL: 47µ; VENDOR: Multicomp; VENDOR-NUMBER: MCCA000491; VOLTAGE: 6,3V
C606 C803 = o.Capacitor 0603 0805 1206; MATERIAL: X7R; ORDER-MULTIPLE: 10; SUPPLIER: Farnell; SUPPLIER-NUMBER: 165-0832; TOLERANCE: 10%; VAL: 10n; VENDOR: Kemet; VENDOR-NUMBER: C0603C103K5RAC; VOLTAGE: 50V
C614 = o.Capacitor 0603 0805 1206; MATERIAL: X7R; ORDER-MULTIPLE: 1; PACKAGE: 1206; PROJECT_LINE1: WordClock; PROJECT_REVISION: 1.05; SUPPLIER: Reichelt; SUPPLIER-NUMBER: X5R-G1206 10/25; TOLERANCE: 10%; VAL: 10µ; VOLTAGE: 25V
C702 C705 C802 = o.Capacitor 0603 0805 1206; MATERIAL: X7R; ORDER-MULTIPLE: 10; SUPPLIER: Farnell; SUPPLIER-NUMBER: 141-4636; TOLERANCE: 10%; VAL: 33n; VENDOR: Kemet; VENDOR-NUMBER: C0603C333K5RAC; VOLTAGE: 50V
C706 C707 = o.Capacitor 0603 0805 1206; MATERIAL: NP0; ORDER-MULTIPLE: 10; SUPPLIER: Farnell; SUPPLIER-NUMBER: 141-4622; TOLERANCE: 5%; VAL: 22p; VENDOR: Kemet; VENDOR-NUMBER: C0603C220J5GAC; VOLTAGE: 50V
C801 = o.Capacitor 0603 0805 1206; MATERIAL: X7R; ORDER-MULTIPLE: 10; SUPPLIER: Farnell; SUPPLIER-NUMBER: 152-0266; TOLERANCE: 10%; VAL: 6n8; VENDOR: Kemet; VENDOR-NUMBER: C0603S682K5RAC; VOLTAGE: 50V
C804 C805 = o.Capacitor 0603 0805 1206; MATERIAL: X7R; ORDER-MULTIPLE: 1; SUPPLIER: Reichelt; SUPPLIER-NUMBER: X7R-G0603 1,5N; TOLERANCE: 10%; VAL: 1n5; VENDOR: YAGEO; VENDOR-NUMBER: 06032R152K9BB0D; VOLTAGE: 50V
D101-D122 D201-D222 D301-D322 D401-D424 D501-D524 = o.Optical.v5; COLOR: White; SUPPLIER: RS Components; SUPPLIER-NUMBER: 664-8226; VAL: LUW T6SG; VENDOR: Osram; VENDOR-NUMBER: LUW T6SG-AABA-4N7Q
D601 = o.Semiconductor.v5; CURRENT: 2A; ORDER-MULTIPLE: 1; SUPPLIER: Farnell; SUPPLIER-NUMBER: 8647836; VAL: 20BQ030; VENDOR: Vishay; VENDOR-NUMBER: 20BQ030PBF; VOLTAGE: 30V
H401 H402 H501 H502 = o.Mechanics
J401 J501 J501A J701 J701A J801 = o.Connectors.v5; SUPPLIER: Reichelt; SUPPLIER-NUMBER: MM FL 4G; VAL: Micro-MaTch 4; VENDOR: Tyco; VENDOR-NUMBER: 0-215079-4
J401A = o.Connectors.v5; PROJECT_LINE1: WordClock; PROJECT_REVISION: 1.05; SUPPLIER: Reichelt; SUPPLIER-NUMBER: MM FL 4G; VAL: Micro-MaTch 4; VENDOR: Tyco; VENDOR-NUMBER: 0-215079-4
J601 = o.Connectors.v5; ORDER-MULTIPLE: 1; SUPPLIER: Farnell; SUPPLIER-NUMBER: 1608727; VAL: PwrJack; VENDOR: Switchcraft; VENDOR-NUMBER: RAPC722X
J602 = o.Connectors.v5; SUPPLIER: Reichelt; SUPPLIER-NUMBER: USB BWM SMD; TYPE: 90° SMD; VAL: USB B-Mini; VENDOR: Assmann; VENDOR-NUMBER: A-USBB-M5/SMD
J603 J604 = o.Connectors.v5; SUPPLIER: Reichelt; SUPPLIER-NUMBER: MM FL 10G; VAL: Micro-MaTch 10; VENDOR: Tyco; VENDOR-NUMBER: 1-215079-0
J702 = o.Connectors.v5; SUPPLIER: Reichelt; SUPPLIER-NUMBER: MM FL 12G; VAL: Micro-MaTch 12; VENDOR: Tyco; VENDOR-NUMBER: 1-215079-2
J703 = o.Connectors.v5; SUPPLIER: Farnell; SUPPLIER-NUMBER: 3418492; VAL: Prog-PDI; VENDOR: Tyco; VENDOR-NUMBER: 826632-3
J704 = o.Connectors.v6; ORDER-MULTIPLE: 1; SUPPLIER: Farnell; SUPPLIER-NUMBER: 1667729; VAL: FTS-105-01-L-DV; VENDOR: Samtec; VENDOR-NUMBER: FTS-105-01-L-DV
L601 = o.Inductor; CURRENT: 180mA; PACKAGE: 0805; RESISTANCE: 2R35; SUPPLIER: Reichelt; SUPPLIER-NUMBER: L-0805AS 1,0µ; TOLERANCE: 5%; VAL: 1µH; VENDOR: FASTRON
MECH801 MECH802 = o.Mechanics; SUPPLIER: Conrad; SUPPLIER-NUMBER: 540387; VAL: KR6G5; VENDOR: Hellermann Tyton; VENDOR-NUMBER: 151-24619
PCB1 = o.PCB Outlines.v6
Q801 = o.Semiconductor.v5; SUPPLIER: Farnell; SUPPLIER-NUMBER: 1081230; VAL: BC847; VENDOR: NXP; VENDOR-NUMBER: BC847
R101-R111 R114-R124 R201-R211 R214-R224 R301-R311 R314-R324 R401-R411 R414-R426 R501-R511 R514-R526 = o.Resistor 0603 0805 1206; ORDER-MULTIPLE: 50; SUPPLIER: DigiKey; SUPPLIER-NUMBER: 541-3.00HCT-ND; TOLERANCE: 1%; VAL: 3R0; VENDOR: Vishay; VENDOR-NUMBER: CRCW06033.00FNEA; WATTAGE: 0,063W
R112 R113 R212 R213 R312 R313 R412 R413 R512 R513 R709 R710 = o.Resistor 0603 0805 1206; ORDER-MULTIPLE: 50; SUPPLIER: Farnell; SUPPLIER-NUMBER: 933-1018; TOLERANCE: 1%; VAL: 330R; VENDOR: multicomp; VENDOR-NUMBER: MC 0.063W 0603 1% 330R; WATTAGE: 0,063W
R601 = o.Resistor 0603 0805 1206; ORDER-MULTIPLE: 50; SUPPLIER: Farnell; SUPPLIER-NUMBER: 933-1360; TOLERANCE: 1%; VAL: 56k; VENDOR: multicomp; VENDOR-NUMBER: MC 0.063W 0603 1% 56k; WATTAGE: 0,063W
R602 R706 R707 = o.Resistor 0603 0805 1206; ORDER-MULTIPLE: 50; SUPPLIER: Farnell; SUPPLIER-NUMBER: 933-1026; TOLERANCE: 1%; VAL: 3k3; VENDOR: multicomp; VENDOR-NUMBER: MC 0.063W 0603 1% 3k3; WATTAGE: 0,063W
R603 = o.Discrete.v6; SUPPLIER: Farnell; SUPPLIER-NUMBER: 514871; TYPE: 3224W; VAL: 1k; VENDOR: Bourns; VENDOR-NUMBER: 3224W-001-102E
R604 R612 = o.Resistor 0603 0805 1206; ORDER-MULTIPLE: 50; SUPPLIER: Farnell; SUPPLIER-NUMBER: 933-0445; TOLERANCE: 1%; VAL: 1k1; VENDOR: multicomp; VENDOR-NUMBER: MC 0.063W 0603 1% 1k1; WATTAGE: 0,063W
R605 R704 R705 R801 = o.Resistor 0603 0805 1206; ORDER-MULTIPLE: 50; SUPPLIER: Farnell; SUPPLIER-NUMBER: 933-0399; TOLERANCE: 1%; VAL: 10k; VENDOR: multicomp; VENDOR-NUMBER: MC 0.063W 0603 1% 10k; WATTAGE: 0,063W
R606 R610 = o.Resistor 0603 0805 1206; ORDER-MULTIPLE: 50; SUPPLIER: Farnell; SUPPLIER-NUMBER: 933-1247; TOLERANCE: 1%; VAL: 4k7; VENDOR: multicomp; VENDOR-NUMBER: MC 0.063W 0603 1% 4k7; WATTAGE: 0,063W
R607 R702 = o.Resistor 0603 0805 1206; ORDER-MULTIPLE: 50; SUPPLIER: Farnell; SUPPLIER-NUMBER: 933-1255; TOLERANCE: 1%; VAL: 47k; VENDOR: multicomp; VENDOR-NUMBER: MC 0.063W 0603 1% 47k; WATTAGE: 0,063W
R608 = o.Resistor 0603 0805 1206; ORDER-MULTIPLE: 50; SUPPLIER: Farnell; SUPPLIER-NUMBER: 933-1034; TOLERANCE: 1%; VAL: 33k; VENDOR: multicomp; VENDOR-NUMBER: MC 0.063W 0603 1% 33k; WATTAGE: 0,063W
R609 = o.Resistor 0603 0805 1206; ORDER-MULTIPLE: 50; SUPPLIER: Farnell; SUPPLIER-NUMBER: 933-0569; TOLERANCE: 1%; VAL: 13k; VENDOR: multicomp; VENDOR-NUMBER: MC 0.063W 0603 1% 13k; WATTAGE: 0,063W
R611 = o.Resistor 0603 0805 1206; ORDER-MULTIPLE: 50; SUPPLIER: Farnell; SUPPLIER-NUMBER: 933-0518; TOLERANCE: 1%; VAL: 12k; VENDOR: multicomp; VENDOR-NUMBER: MC 0.063W 0603 1% 12k; WATTAGE: 0,063W
R701 R703 R802 = o.Resistor 0603 0805 1206; ORDER-MULTIPLE: 50; SUPPLIER: Farnell; SUPPLIER-NUMBER: 933-0364; TOLERANCE: 1%; VAL: 100R; VENDOR: multicomp; VENDOR-NUMBER: MC 0.063W 0603 1% 100R; WATTAGE: 0,063W
R708 = o.Discrete.v6; SUPPLIER: Reichelt; SUPPLIER-NUMBER: LDR 07; VAL: A906009; VENDOR: PerkinElmer; VENDOR-NUMBER: A 9060 09
R708A R708B = o.Discrete.v6; PROJECT_LINE1: WordClock; PROJECT_REVISION: 1.05; SUPPLIER: Reichelt; SUPPLIER-NUMBER: LDR 07; VAL: A906009; VENDOR: PerkinElmer; VENDOR-NUMBER: A 9060 09
R803 = o.Resistor 0603 0805 1206; ORDER-MULTIPLE: 50; SUPPLIER: Farnell; SUPPLIER-NUMBER: 933-0402; TOLERANCE: 1%; VAL: 100k; VENDOR: multicomp; VENDOR-NUMBER: MC 0.063W 0603 1% 100k; WATTAGE: 0,063W
U101 U201 U301 U401 U501 = o.Semiconductor.v5; SUPPLIER: DigiKey; SUPPLIER-NUMBER: 568-4774-1-ND; VAL: PCA9626B; VENDOR: NXP; VENDOR-NUMBER: PCA9626B
U601 U603 = o.Semiconductor.v5; IOUT: 3A; ORDER-MULTIPLE: 1; SUPPLIER: DigiKey; SUPPLIER-NUMBER: LMZ12003TZ-ADJCT-ND; VAL: LMZ12003; VENDOR: National Semiconductor; VENDOR-NUMBER: LMZ12003 TZ-ADJ; VIN: 4,5 -20V; VOUT: 0,8 - 6V
U602 = o.Controller.v5; SUPPLIER: Reichelt; SUPPLIER-NUMBER: FT 232 RL; VAL: FT232RL; VENDOR: FTDI Chip; VENDOR-NUMBER: FT232RL
U701 = o.Semiconductor.v5; SUPPLIER: Reichelt; SUPPLIER-NUMBER: LHI 1128; VAL: LHi 1128; VENDOR: PerkinElmer; VENDOR-NUMBER: LHi 1128
U702 = o.Semiconductor.v5; SUPPLIER: Farnell; SUPPLIER-NUMBER: 4913103; VAL: TSOP32236; VENDOR: Vishay; VENDOR-NUMBER: TSOP32236
U703 = o.Semiconductor.v5; SUPPLIER: Farnell; SUPPLIER-NUMBER: 1292233; VAL: MCP120-300; VENDOR: Microchip; VENDOR-NUMBER: MCP120-300I/TT
U704 = o.Controller.v5; EEPROM: 2k; FLASH: 64k + 4k; SRAM: 4k; SUPPLIER: Farnell; SUPPLIER-NUMBER: 1748559; VAL: ATxmega64A3-AU; VENDOR: Atmel; VENDOR-NUMBER: ATxmega64A3-AU
U801 = o.Semiconductor.v5; SUPPLIER: www.electronicpool.de; SUPPLIER-NUMBER: U4224B; VAL: U4224B; VENDOR: Temic; VENDOR-NUMBER: U4224B
X1-X18 X21-X24 X401-X404 X501-X504 X801 X802 = o.Connectors.v5
XTAL701 = o.Crystal.v5; SUPPLIER: Reichelt; SUPPLIER-NUMBER: 8,000000-MQ; VAL: 8,0MHz; VENDOR: Euroquartz; VENDOR-NUMBER: 8.000MHz MQ/30/30/40/12pF/60R
XTAL801 XTAL802 = o.Crystal.v5; SUPPLIER: Conrad; SUPPLIER-NUMBER: 168432-62; VAL: 77.5kHz; VENDOR: n/a; VENDOR-NUMBER: n/a

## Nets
12V0: C602.1 C611.1 C614.1 D601.C J604.1 J604.2 J604.3 R601.1 R607.1 R608.1 U601.1 U603.1
+3V3: C103.1 C104.1 C203.1 C204.1 C303.1 C304.1 C403.1 C404.1 C503.1 C504.1 C605.1 C613.1 C704.1 C708.1 C709.1 C710.1 C711.1 C712.1 C713.1 C714.1 J604.9 J604.10 J701.4 J701A.4 J702.3 J703.2 J704.4 R609.1 R610.1 R701.1 R703.1 R704.1 R705.1 R706.1 R707.1 U101.23 U101.40 U201.23 U201.40 U201.46 U301.23 U301.40 U301.47 U401.23 U401.40 U401.46 U401.47 U501.13 U501.23 U501.40 U603.7 U703.2 U704.15 U704.25 U704.35 U704.45 U704.53 U704.61 X23.P$1 X24.P$1
+3V3A: C609.1 J603.9 J603.10 U602.4
D+: J602.3 U602.15
D-: J602.2 U602.16
DCF77#: J701.2 J701A.2 U704.7
DISP-A0: J702.2 U704.18
DISP-CLK: J702.7 U704.23
DISP-CS#: J702.5 U704.20
DISP-DIN: J702.6 U704.21
DISP-RESET#: J702.4 U704.19
GND: C101.2 C102.2 C103.2 C104.2 C105.2 C106.2 C201.2 C202.2 C203.2 C204.2 C205.2 C206.2 C301.2 C302.2 C303.2 C304.2 C305.2 C306.2 C401.2 C402.2 C403.2 C404.2 C405.2 C406.2 C501.2 C502.2 C503.2 C504.2 C505.2 C506.2 C602.2 C603.2 C604.2 C611.2 C612.2 C613.2 C614.2 C615.2 C701.2 C702.2 C703.2 C704.2 C705.2 C706.2 C707.2 C708.2 C709.2 C710.2 C711.2 C712.2 C713.2 C714.2 D601.A J604.4 J604.6 J604.8 J701.1 J701A.1 J702.1 J702.12 J703.6 J704.2 J704.10 R604.2 R611.2 R612.2 R702.2 R708.2 R708A.2 R708B.2 U101.1 U101.6 U101.7 U101.12 U101.13 U101.14 U101.15 U101.16 U101.21 U101.22 U101.25 U101.30 U101.31 U101.36 U101.37 U101.45 U101.46 U101.47 U101.48 U201.1 U201.6 U201.7 U201.12 U201.13 U201.14 U201.15 U201.16 U201.21 U201.22 U201.25 U201.30 U201.31 U201.36 U201.37 U201.45 U201.47 U201.48 U301.1 U301.6 U301.7 U301.12 U301.13 U301.14 U301.15 U301.16 U301.21 U301.22 U301.25 U301.30 U301.31 U301.36 U301.37 U301.45 U301.46 U301.48 U401.1 U401.6 U401.7 U401.12 U401.13 U401.14 U401.15 U401.16 U401.21 U401.22 U401.25 U401.30 U401.31 U401.36 U401.37 U401.45 U401.48 U501.1 U501.6 U501.7 U501.12 U501.14 U501.15 U501.16 U501.21 U501.22 U501.25 U501.30 U501.31 U501.36 U501.37 U501.45 U501.46 U501.47 U501.48 U601.4 U601.HS U603.4 U603.HS U701.3 U702.3 U703.3 U704.14 U704.24 U704.34 U704.44 U704.52 U704.60 X21.P$1 X22.P$1
GND1: C806.2 C807.2 C808.2 J801.1 Q801.2 U801.3 U801.4
GNDA: C606.2 C607.2 C608.2 C609.2 C610.2 J601.2 J601.3 J602.5 J602.S0 J602.S1 J602.S2 J602.S3 J603.4 J603.6 J603.8 R605.1 U602.7 U602.18 U602.21 U602.25 U602.26
IR: U702.1 U704.64
KEY0: J702.8 U704.30
KEY1: J702.9 U704.31
KEY2: J702.10 U704.32
KEY3: J702.11 U704.33
LDR: C705.1 R705.2 R708.1 R708A.1 R708B.1 U704.63
LED0@U1: D101.C U101.2
LED0@U2: D201.C U201.2
LED0@U3: D301.C U301.2
LED0@U4: D401.C U401.2
LED0@U5: D501.C U501.2
LED1@U1: D102.C U101.3
LED1@U2: D202.C U201.3
LED1@U3: D302.C U301.3
LED1@U4: D402.C U401.3
LED1@U5: D502.C U501.3
LED2@U1: D103.C U101.4
LED2@U2: D203.C U201.4
LED2@U3: D303.C U301.4
LED2@U4: D403.C U401.4
LED2@U5: D503.C U501.4
LED3@U1: D104.C U101.5
LED3@U2: D204.C U201.5
LED3@U3: D304.C U301.5
LED3@U4: D404.C U401.5
LED3@U5: D504.C U501.5
LED4@U1: D105.C U101.8
LED4@U2: D205.C U201.8
LED4@U3: D305.C U301.8
LED4@U4: D405.C U401.8
LED4@U5: D505.C U501.8
LED5@U1: D106.C U101.9
LED5@U2: D206.C U201.9
LED5@U3: D306.C U301.9
LED5@U4: D406.C U401.9
LED5@U5: D506.C U501.9
LED6@U1: D107.C U101.10
LED6@U2: D207.C U201.10
LED6@U3: D307.C U301.10
LED6@U4: D407.C U401.10
LED6@U5: D507.C U501.10
LED7@U1: D108.C U101.11
LED7@U2: D208.C U201.11
LED7@U3: D308.C U301.11
LED7@U4: D408.C U401.11
LED7@U5: D508.C U501.11
LED8@U1: D109.C U101.17
LED8@U2: D209.C U201.17
LED8@U3: D309.C U301.17
LED8@U4: D409.C U401.17
LED8@U5: D509.C U501.17
LED9@U1: D110.C U101.18
LED9@U2: D210.C U201.18
LED9@U3: D310.C U301.18
LED9@U4: D410.C U401.18
LED9@U5: D510.C U501.18
LED10@U1: D111.C U101.19
LED10@U2: D211.C U201.19
LED10@U3: D311.C U301.19
LED10@U4: D411.C U401.19
LED10@U5: D511.C U501.19
LED11@U1: D122.C U101.20
LED11@U2: D222.C U201.20
LED11@U3: D322.C U301.20
LED11@U4: D422.C U401.20
LED11@U5: D522.C U501.20
LED12@U1: D121.C U101.26
LED12@U2: D221.C U201.26
LED12@U3: D321.C U301.26
LED12@U4: D421.C U401.26
LED12@U5: D521.C U501.26
LED13@U1: D120.C U101.27
LED13@U2: D220.C U201.27
LED13@U3: D320.C U301.27
LED13@U4: D420.C U401.27
LED13@U5: D520.C U501.27
LED14@U1: D119.C U101.28
LED14@U2: D219.C U201.28
LED14@U3: D319.C U301.28
LED14@U4: D419.C U401.28
LED14@U5: D519.C U501.28
LED15@U1: D118.C U101.29
LED15@U2: D218.C U201.29
LED15@U3: D318.C U301.29
LED15@U4: D418.C U401.29
LED15@U5: D518.C U501.29
LED16@U1: D117.C U101.32
LED16@U2: D217.C U201.32
LED16@U3: D317.C U301.32
LED16@U4: D417.C U401.32
LED16@U5: D517.C U501.32
LED17@U1: D116.C U101.33
LED17@U2: D216.C U201.33
LED17@U3: D316.C U301.33
LED17@U4: D416.C U401.33
LED17@U5: D516.C U501.33
LED18@U1: D115.C U101.34
LED18@U2: D215.C U201.34
LED18@U3: D315.C U301.34
LED18@U4: D415.C U401.34
LED18@U5: D515.C U501.34
LED19@U1: D114.C U101.35
LED19@U2: D214.C U201.35
LED19@U3: D314.C U301.35
LED19@U4: D414.C U401.35
LED19@U5: D514.C U501.35
LED20@U1: D113.C U101.41
LED20@U2: D213.C U201.41
LED20@U3: D313.C U301.41
LED20@U4: D413.C U401.41
LED20@U5: D513.C U501.41
LED21@U1: D112.C U101.42
LED21@U2: D212.C U201.42
LED21@U3: D312.C U301.42
LED21@U4: D412.C U401.42
LED21@U5: D512.C U501.42
MATRIX-OE#: U101.24 U201.24 U301.24 U401.24 U501.24 U704.55
MATRIX-PWR: U601.3 U704.9
MATRIX-SCL: R113.1 R213.1 R313.1 R413.1 R513.1 R706.2 R710.1
MATRIX-SDA: R112.1 R212.1 R312.1 R412.1 R512.1 R707.2 R709.1
N$1: R709.2 U704.16
N$2: R710.2 U704.17
N$3: R608.2 R611.1 U603.3
N$4: C605.2 R609.2 R610.2 R612.1 U603.6
N$5: C601.2 R603.2 R603.3 R604.1 U601.6
N$6: C603.1 U601.5
N$7: R601.2 U601.2
N$8: C612.1 U603.5
N$9: J703.1 U704.56
N$10: R607.2 U603.2
N$11: J703.5 J704.6 R704.2 U703.1 U704.57
N$12: C707.1 U704.59 XTAL701.3
N$13: C706.1 U704.58 XTAL701.1
N$14: C610.1 U602.17
N$15: C607.1 C608.1 L601.2 R606.1 U602.20
N$16: U801.5 XTAL801.2
N$19: D523.C X503.1
N$20: U801.6 XTAL801.1
N$21: U801.13 XTAL802.2
N$22: U801.14 XTAL802.1
N$23: C804.1 C805.1 C806.1 C807.1 R802.1 U801.1 U801.12 X801.1
N$24: C808.1 J801.4 R801.1 R802.2
N$25: C801.1 U801.7
N$26: C801.2 C802.1 U801.8
N$27: C802.2 U801.9
N$28: C803.1 U801.10
N$29: C803.2 U801.11
N$30: J801.3 U801.15
N$31: C804.2 C805.2 U801.2 X802.1
N$32: J801.2 Q801.3 R801.2
N$33: Q801.1 R803.2
N$34: R803.1 U801.16
N$36: C701.1 R701.2 U701.1
N$38: J501.2 J501A.2 U501.43
N$39: C703.1 R703.2 U702.2
N$40: D523.A R525.2
N$41: J501.4 J501A.4 U501.44
N$42: R525.1 X501.1
N$44: R526.1 X502.1
N$45: D524.C X504.1
N$46: D524.A R526.2
N$48: J401.2 J401A.2 U401.43
N$54: J401.4 J401A.4 U401.44
N$55: D423.C X403.1
N$56: D423.A R425.2
N$57: R425.1 X401.1
N$58: R426.1 X402.1
N$60: D424.C X404.1
N$62: D424.A R426.2
N$69: J601.1 J603.1 J603.2 J603.3
N$70: J603.5 U602.1
N$71: J603.7 U602.5
N$73: R602.2 R603.1
N$87: C606.1 J602.1 L601.1
N$88: R605.2 R606.2 U602.19
PA3: U704.1 X9.P$1
PA4: U704.2 X10.P$1
PA5: U704.3 X11.P$1
PA6: U704.4 X12.P$1
PA7: U704.5 X13.P$1
PB0: U704.6 X14.P$1
PB4: J704.5 U704.10 X15.P$1
PB5: J704.9 U704.11 X16.P$1
PB6: J704.1 U704.12 X17.P$1
PB7: J704.3 U704.13 X18.P$1
PE0: U704.36 X1.P$1
PE1: U704.37 X2.P$1
PE2: U704.38 X3.P$1
PE3: U704.39 X4.P$1
PE4: U704.40 X5.P$1
PE5: U704.41 X6.P$1
PE6: U704.42 X7.P$1
PE7: U704.43 X8.P$1
PIR: C702.1 R702.1 U701.2 U704.62
R1@U1: D101.A R101.2
R1@U2: D201.A R201.2
R1@U3: D301.A R301.2
R1@U4: D401.A R401.2
R1@U5: D501.A R501.2
R2@U1: D102.A R102.2
R2@U2: D202.A R202.2
R2@U3: D302.A R302.2
R2@U4: D402.A R402.2
R2@U5: D502.A R502.2
R3@U1: D103.A R103.2
R3@U2: D203.A R203.2
R3@U3: D303.A R303.2
R3@U4: D403.A R403.2
R3@U5: D503.A R503.2
R4@U1: D104.A R104.2
R4@U2: D204.A R204.2
R4@U3: D304.A R304.2
R4@U4: D404.A R404.2
R4@U5: D504.A R504.2
R5@U1: D105.A R105.2
R5@U2: D205.A R205.2
R5@U3: D305.A R305.2
R5@U4: D405.A R405.2
R5@U5: D505.A R505.2
R6@U1: D106.A R106.2
R6@U2: D206.A R206.2
R6@U3: D306.A R306.2
R6@U4: D406.A R406.2
R6@U5: D506.A R506.2
R7@U1: D107.A R107.2
R7@U2: D207.A R207.2
R7@U3: D307.A R307.2
R7@U4: D407.A R407.2
R7@U5: D507.A R507.2
R8@U1: D108.A R108.2
R8@U2: D208.A R208.2
R8@U3: D308.A R308.2
R8@U4: D408.A R408.2
R8@U5: D508.A R508.2
R9@U1: D109.A R109.2
R9@U2: D209.A R209.2
R9@U3: D309.A R309.2
R9@U4: D409.A R409.2
R9@U5: D509.A R509.2
R10@U1: D110.A R110.2
R10@U2: D210.A R210.2
R10@U3: D310.A R310.2
R10@U4: D410.A R410.2
R10@U5: D510.A R510.2
R11@U1: D111.A R111.2
R11@U2: D211.A R211.2
R11@U3: D311.A R311.2
R11@U4: D411.A R411.2
R11@U5: D511.A R511.2
R12@U1: D112.A R114.1
R12@U2: D212.A R214.1
R12@U3: D312.A R314.1
R12@U4: D412.A R414.1
R12@U5: D512.A R514.1
R13@U1: D113.A R115.1
R13@U2: D213.A R215.1
R13@U3: D313.A R315.1
R13@U4: D413.A R415.1
R13@U5: D513.A R515.1
R14@U1: D114.A R116.1
R14@U2: D214.A R216.1
R14@U3: D314.A R316.1
R14@U4: D414.A R416.1
R14@U5: D514.A R516.1
R15@U1: D115.A R117.1
R15@U2: D215.A R217.1
R15@U3: D315.A R317.1
R15@U4: D415.A R417.1
R15@U5: D515.A R517.1
R16@U1: D116.A R118.1
R16@U2: D216.A R218.1
R16@U3: D316.A R318.1
R16@U4: D416.A R418.1
R16@U5: D516.A R518.1
R17@U1: D117.A R119.1
R17@U2: D217.A R219.1
R17@U3: D317.A R319.1
R17@U4: D417.A R419.1
R17@U5: D517.A R519.1
R18@U1: D118.A R120.1
R18@U2: D218.A R220.1
R18@U3: D318.A R320.1
R18@U4: D418.A R420.1
R18@U5: D518.A R520.1
R19@U1: D119.A R121.1
R19@U2: D219.A R221.1
R19@U3: D319.A R321.1
R19@U4: D419.A R421.1
R19@U5: D519.A R521.1
R20@U1: D120.A R122.1
R20@U2: D220.A R222.1
R20@U3: D320.A R322.1
R20@U4: D420.A R422.1
R20@U5: D520.A R522.1
R21@U1: D121.A R123.1
R21@U2: D221.A R223.1
R21@U3: D321.A R323.1
R21@U4: D421.A R423.1
R21@U5: D521.A R523.1
R22@U1: D122.A R124.1
R22@U2: D222.A R224.1
R22@U3: D322.A R324.1
R22@U4: D422.A R424.1
R22@U5: D522.A R524.1
RCV-EN#: J701.3 J701A.3 U704.8
RXD: J604.7 U704.49
SCL@U1: R113.2 U101.38
SCL@U2: R213.2 U201.38
SCL@U3: R313.2 U301.38
SCL@U4: R413.2 U401.38
SCL@U5: R513.2 U501.38
SDA@U1: R112.2 U101.39
SDA@U2: R212.2 U201.39
SDA@U3: R312.2 U301.39
SDA@U4: R412.2 U401.39
SDA@U5: R512.2 U501.39
TXD: J604.5 U704.48
V+: C101.1 C102.1 C105.1 C106.1 C201.1 C202.1 C205.1 C206.1 C301.1 C302.1 C305.1 C306.1 C401.1 C402.1 C405.1 C406.1 C501.1 C502.1 C505.1 C506.1 C601.1 C604.1 C615.1 J401.1 J401.3 J401A.1 J401A.3 J501.1 J501.3 J501A.1 J501A.3 R101.1 R102.1 R103.1 R104.1 R105.1 R106.1 R107.1 R108.1 R109.1 R110.1 R111.1 R114.2 R115.2 R116.2 R117.2 R118.2 R119.2 R120.2 R121.2 R122.2 R123.2 R124.2 R201.1 R202.1 R203.1 R204.1 R205.1 R206.1 R207.1 R208.1 R209.1 R210.1 R211.1 R214.2 R215.2 R216.2 R217.2 R218.2 R219.2 R220.2 R221.2 R222.2 R223.2 R224.2 R301.1 R302.1 R303.1 R304.1 R305.1 R306.1 R307.1 R308.1 R309.1 R310.1 R311.1 R314.2 R315.2 R316.2 R317.2 R318.2 R319.2 R320.2 R321.2 R322.2 R323.2 R324.2 R401.1 R402.1 R403.1 R404.1 R405.1 R406.1 R407.1 R408.1 R409.1 R410.1 R411.1 R414.2 R415.2 R416.2 R417.2 R418.2 R419.2 R420.2 R421.2 R422.2 R423.2 R424.2 R501.1 R502.1 R503.1 R504.1 R505.1 R506.1 R507.1 R508.1 R509.1 R510.1 R511.1 R514.2 R515.2 R516.2 R517.2 R518.2 R519.2 R520.2 R521.2 R522.2 R523.2 R524.2 R602.1 U601.7

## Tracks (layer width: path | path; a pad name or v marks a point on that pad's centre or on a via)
12V0  (via drill 0.5)
  Top 0.406: 244.71,7.53 244.33,7.53 U603.1 | 249.7,4.61 R608.1 | 249.7,4.61 R607.1 | C611.1 249.7,4.61 | R601.1 277.98,15.28 U601.1
  Top 0.61: 265.15,5.12 J604.2 | 265.15,5.12 J604.3 | 265.15,5.12 J604.1 D601.C 273.7,20.36 C614.1 C602.1 277.98,15.28 | v244.71,2.58 C611.1
  Top 0.813: C611.1
  Top 1.016: C611.1 244.71,7.53
  Bottom 0.61: J604.2 263.88,1.31 254.23,1.31 252.96,2.58 v244.71,2.58
+3V3  (via drill 0.5, 0.6)
  Top 0.254: v140.74,301.16 144.76,301.16 v146.26,299.65 | v146.26,237.65 144.76,239.16 v140.74,239.16 v140.74,241.59 | v146.26,175.65 144.76,177.16 v140.74,177.16 v140.74,180.13 | v146.26,113.65 144.76,115.16 v140.74,115.16 v140.74,116.91 | v140.74,53.16 144.76,53.16 | 144.76,53.16 v146.26,51.65 | v146.25,56.66 146.25,54.66 144.76,53.16 | X24.P$1 X23.P$1 241.53,24.68
  Top 0.406: C605.1 R610.1 R609.1 252.96,16.3 253.59,16.93 253.59,19.09 252.71,19.98 248.51,19.98 246.86,18.33 C613.1 | 244.71,15.66 244.59,15.66 U603.7 | v220.57,41.87 220.55,41.9 | 224.16,44.47 v224.18,44.49 | v264.52,69.89 254.23,69.89 v245.34,61 | J703.2 263.75,15.79 263.75,21.38
  Top 0.61: v131.04,233.72 v136.12,233.72 | v131.04,171.74 v135.87,171.74 | v131.04,109.77 v135.87,109.77 | v131.04,47.66 v135.87,47.66 | 254.99,21.38 263.75,21.38 276.58,21.38 276.96,21.76 v285.73,21.76 v300.84,21.76 | 254.99,21.38 v247.88,21.38 244.71,21.38 | v235.16,30.82 234.37,30.82 232.78,32.41 | 230.66,41.87 v230.66,44.49 230.66,44.5 | 224.16,41.87 224.16,44.47 | 224.16,41.87 v220.57,41.87 | 230.66,41.87 224.16,41.87 | 232.78,32.41 230.66,34.53 | 230.66,34.53 230.66,41.87 | v220.57,33.85 221.26,34.53 226.42,34.53 | 230.66,34.53 226.42,34.53 | 226.42,34.53 v226.42,31.79 | 232.78,32.41 v233.28,32.88 | 254.99,21.38 254.99,5.12 | 254.99,5.12 J604.10 | 254.99,5.12 J604.9
  Top 1.016: v131.04,295.82 v136.65,295.82 | v131.04,24.68 v163.43,24.68 v198.96,24.68 v236.58,24.68 | v236.58,24.68 241.53,24.68 242.67,24.68 244.71,22.65 244.71,21.38 C613.1 244.71,15.66 | v236.58,24.68 236.58,23.23 234.88,21.53 228.73,21.53 v225.02,17.82
  Bottom 0.254: 138.15,300.52 138.28,300.65 U101.40 140.24,300.65 v140.74,301.16 | v146.26,299.65 U101.23 | 138.15,238.52 138.28,238.65 U201.40 140.24,238.65 v140.74,239.16 | v146.26,237.65 U201.23 | 138.15,176.52 138.28,176.65 U301.40 140.24,176.65 v140.74,177.16 | v146.26,175.65 U301.23 | 138.15,114.52 138.28,114.65 U401.40 140.24,114.65 v140.74,115.16 | v146.26,113.65 U401.23 | 138.15,52.52 138.28,52.65 U501.40 140.24,52.65 v140.74,53.16 | v146.26,51.65 U501.23 | U501.13 146.51,56.65 v146.25,56.66 | U401.47 140.49,118.15 140.74,117.9 140.74,117.65 | v140.74,180.13 140.67,180.15 U301.47 | U201.46 140.64,241.65 v140.74,241.59 | R704.1 215.11,50.84 214.22,49.95 211.94,49.95 211.12,50.77 U703.2 | 198.96,53.13 198.99,53.1 | 198.96,51.09 198.99,51.07 | 140.74,117.65 U401.46 | v140.74,116.91 140.74,117.65 | J704.4 248.51,25.44 247.88,24.8 v247.88,21.38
